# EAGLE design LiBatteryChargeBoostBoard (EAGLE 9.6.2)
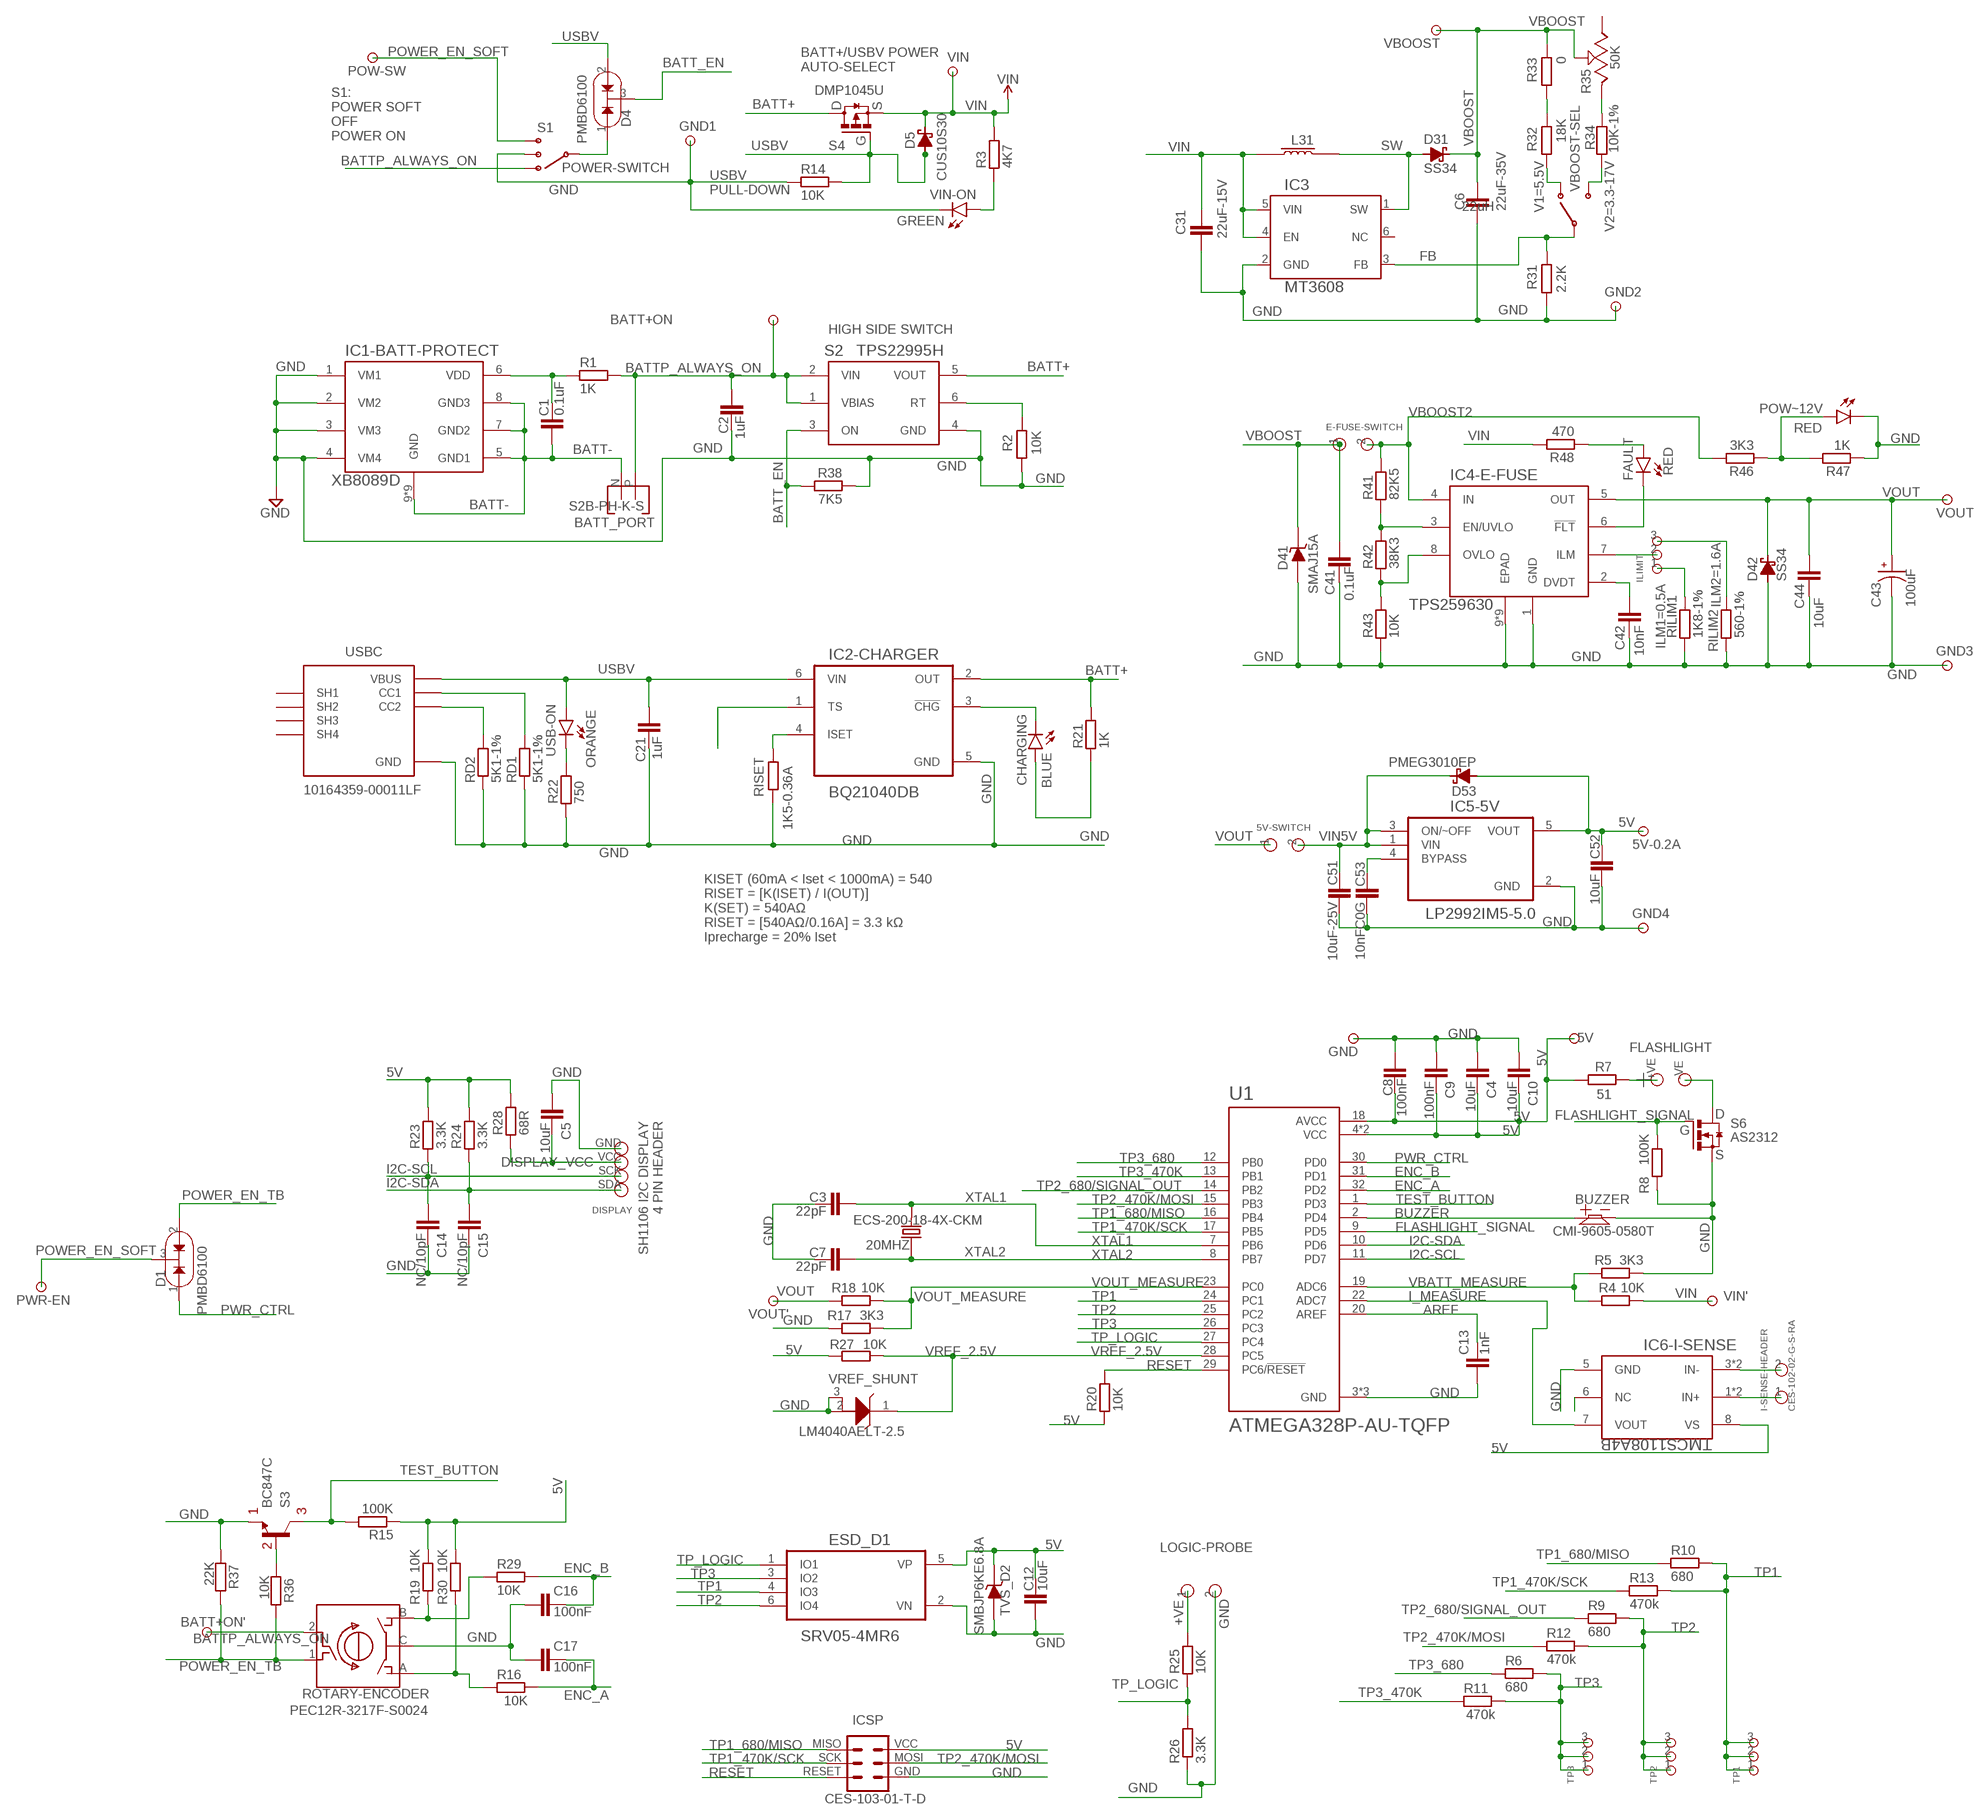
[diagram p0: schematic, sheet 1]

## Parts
5V  TEST-POINT-TH  [TEST-POINT-TH-1MM]
5V-0.2A  TEST-POINT-TH  [TEST-POINT-TH-1MM]
5V-SWITCH  HEADER-2PIN-0.1"P  [HEADER-2PIN-0.1"P]
20MHZ  ECS-200-18-4X-CKM  CRYSTAL-20MHZ-ECS-200-18-4X-CKM  [XTAL_ECS-200-18-4X-CKM]
BATT+ON  TEST-POINT-TH  [TEST-POINT-TH-1MM]
BATT+ON'  TEST-POINT-TH  [TEST-POINT-TH-1MM]
BATT_PORT  S2B-PH-K-S  [S2B-PH-K-S]
BUZZER  CMI-9605-0580T  BUZZER-ACTIVE-CMI-9605-0580T  [BUZZER-ACTIVE-CMI-9605-0580T]
C1  0.1uF  CAPACITOR_SMD0603  [0603]
C2  1uF  CAPACITOR_SMD0603  [0603]
C3  22pF  CAPACITOR_SMD0603  [0603]
C4  10uF  CAPACITOR_SMD0603  [0603]
C5  10uF  CAPACITOR1206  [1206]
C6  22uF-35V  CAPACITOR_SMD1206  [1206]
C7  22pF  CAPACITOR_SMD0603  [0603]
C8  100nF  CAPACITOR_SMD0603  [0603]
C9  100nF  CAPACITOR_SMD0603  [0603]
C10  10uF  CAPACITOR_SMD0603  [0603]
C12  10uF  CAPACITOR_SMD0603  [0603]
C13  1nF  CAPACITOR_SMD0603  [0603]
C14  NC/10pF  CAPACITOR_SMD0603  [0603]
C15  NC/10pF  CAPACITOR_SMD0603  [0603]
C16  100nF  CAPACITOR_SMD0603  [0603]
C17  100nF  CAPACITOR_SMD0603  [0603]
C21  1uF  CAPACITOR_SMD0603  [0603]
C31  22uF-15V  CAPACITOR_SMD1206  [1206]
C41  0.1uF  CAPACITOR_SMD0603  [0603]
C42  10nF  CAPACITOR_SMD0603  [0603]
C43  100uF  EEEFN1E101UP  [CAP_EEEFN1E101UP]
C44  10uF  CAPACITOR_SMD0603  [0603]
C51  10uF-25V  CAPACITOR0603  [0603]
C52  10uF  CAPACITOR0603  [0603]
C53  10nFC0G  CAPACITOR_SMD0603  [0603]
CHARGING  BLUE  LED0603  [0603-DIODE]
D1  PMBD6100  DIODE-DOUBLE-COMMON-CATHODE-PMBD6100,215  [SOT-23-3]
D4  PMBD6100  DIODE-DOUBLE-COMMON-CATHODE-PMBD6100,215  [SOT-23-3]
D5  CUS10S30  DIODE-SCHOTTKY-CUS10S30,H3F  [SOD-323]
D31  SS34  DIODE-SCHOTTKY-SS34  [SMA]
D41  SMAJ15A  DIODE-TVS-SMA  [SMA]
D42  SS34  DIODE-SCHOTTKY-SS34  [SMA]
D53  PMEG3010EP  DIODE-SCHOTTKY-PMEG3010EP,115  [SOD-128]
DISPLAY  DISPLAY-1.3"-SH1106-I2C  [DISPLAY-1.3"-SH1106-I2C]
E-FUSE-SWITCH  HEADER-2PIN-0.1"P  [HEADER-2PIN-0.1"P]
ESD_D1  SRV05-4MR6  SRV05-4MR6T1G  [SOT-23-6]
FAULT  RED  LED0603  [0603-DIODE]
FLASHLIGHT  HEADER-2PIN-0.2"P  [HEADER-2PIN-0.2"P]
GND  TEST-POINT-TH  [TEST-POINT-TH-1MM]
GND1  TEST-POINT-TH  [TEST-POINT-TH-1MM]
GND2  TEST-POINT-TH  [TEST-POINT-TH-1MM]
GND3  TEST-POINT-TH  [TEST-POINT-TH-1MM]
GND4  TEST-POINT-TH  [TEST-POINT-TH-1MM]
I-SENSE-HEADER  CES-102-02-G-S-RA  HEADER-2PIN-0.1"P  [HEADER-2PIN-0.1"P]
IC1-BATT-PROTECT  XB8089D  [SOIC-8-POWER-PAD]
IC2-CHARGER  BQ21040DB  BQ21040DBVR  [SOT-23-6]
IC3  MT3608  [SOT-23-6]
IC4-E-FUSE  TPS259630  TPS259621DDAR  [SOIC-8-POWER-PAD]
IC5-5V  LP2992IM5-5.0  [SOT-23-5]
IC6-I-SENSE  TMCS1108A4B  TMCS1108A4B-CURRENT-SENSE  [SOIC-8]
ICSP  CES-103-01-T-D  HEADER-ICSP-0.1"P  [HEADER-ICSP-0.1"P]
ILIMIT  HEADER-3PIN-0.1"P  [HEADER-3PIN-0.1"P]
L31  22uH  INDUCTOR-SMRH74-220MT  [INDUCTOR-SMRH74-220MT]
LOGIC-PROBE  HEADER-2PIN-0.1"P  [HEADER-2PIN-0.1"P]
POW-SW  TEST-POINT-TH  [TEST-POINT-TH-1MM]
POW~12V  RED  LED1206  [1206-DIODE]
PWR-EN  TEST-POINT-TH  [TEST-POINT-TH-1MM]
R1  1K  RESISTOR_SMD0603  [0603]
R2  10K  RESISTOR_SMD0603  [0603]
R3  4K7  RESISTOR_SMD0603  [0603]
R4  10K  RESISTOR_SMD0603  [0603]
R5  3K3  RESISTOR_SMD0603  [0603]
R6  680  RESISTOR_SMD1206  [1206]
R7  51  RESISTOR_SMD1206  [1206]
R8  100K  RESISTOR_SMD0603  [0603]
R9  680  RESISTOR_SMD1206  [1206]
R10  680  RESISTOR_SMD1206  [1206]
R11  470k  RESISTOR_SMD1206  [1206]
R12  470k  RESISTOR_SMD1206  [1206]
R13  470k  RESISTOR_SMD1206  [1206]
R14  10K  RESISTOR_SMD0603  [0603]
R15  100K  RESISTOR_SMD0603  [0603]
R16  10K  RESISTOR_SMD0603  [0603]
R17  3K3  RESISTOR_SMD0603  [0603]
R18  10K  RESISTOR_SMD0603  [0603]
R19  10K  RESISTOR_SMD0603  [0603]
R20  10K  RESISTOR_SMD0603  [0603]
R21  1K  RESISTOR_SMD0603  [0603]
R22  750  RESISTOR_SMD0603  [0603]
R23  3.3K  RESISTOR_SMD0603  [0603]
R24  3.3K  RESISTOR_SMD0603  [0603]
R25  10K  RESISTOR_SMD0603  [0603]
R26  3.3K  RESISTOR_SMD0603  [0603]
R27  10K  RESISTOR_SMD0603  [0603]
R28  68R  RESISTOR_SMD0603  [0603]
R29  10K  RESISTOR_SMD0603  [0603]
R30  10K  RESISTOR_SMD0603  [0603]
R31  2.2K  RESISTOR_SMD0603  [0603]
R32  18K  RESISTOR_SMD0603  [0603]
R33  0  RESISTOR_SMD0603  [0603]
R34  10K-1%  RESISTOR_SMD0603  [0603]
R35  50K  ROTARY-POTENTIOMETER-3386P-1-503TLF  [ROTARY-POTENTIOMETER-3386P]
R36  10K  RESISTOR_SMD0603  [0603]
R37  22K  RESISTOR_SMD0603  [0603]
R38  7K5  RESISTOR_SMD0603  [0603]
R41  82K5  RESISTOR_SMD0603  [0603]
R42  38K3  RESISTOR_SMD0603  [0603]
R43  10K  RESISTOR_SMD0603  [0603]
R46  3K3  RESISTOR_SMD0603  [0603]
R47  1K  RESISTOR_SMD0603  [0603]
R48  470  RESISTOR_SMD0603  [0603]
RD1  5K1-1%  RESISTOR_SMD0603  [0603]
RD2  5K1-1%  RESISTOR_SMD0603  [0603]
RILIM1  1K8-1%  RESISTOR_SMD0603  [0603]
RILIM2  560-1%  RESISTOR_SMD0603  [0603]
RISET  1K5-0.36A  RESISTOR_SMD0603  [0603]
ROTARY-ENCODER  PEC12R-3217F-S0024  [PEC12R-3217F-S0024]
S1  POWER-SWITCH  SLIDE-SWITCH-SP3T-VER-TH-MINI  [CSS-1310MC]
S2  TPS22995H  TPS22995H-Q1  [SOT-23-6]
S3  BC847C  [SOT-23-3]
S4  DMP1045U  [SOT-23-3]
S6  AS2312  AS2312AS2312  [SOT-23-3]
TP1  HEADER-3PIN-0.1"P  [HEADER-3PIN-0.1"P]
TP2  HEADER-3PIN-0.1"P  [HEADER-3PIN-0.1"P]
TP3  HEADER-3PIN-0.1"P  [HEADER-3PIN-0.1"P]
TVS_D2  SMBJP6KE6.8A  SMBJP6KE6.8A-TP  [DIOM5336X244N]
U1  ATMEGA328P-AU-TQFP  [TQFP32]
USB-ON  ORANGE  LED0603  [0603-DIODE]
USBC  10164359-00011LF  USB-C-RECEPTABLE-10164359-00011LF  [USB-C-RECEPTABLE-1016435900011LF]
VBOOST  TEST-POINT-TH  [TEST-POINT-TH-1MM]
VBOOST-SEL  SLIDE-SWITCH-SPDT-VERTICLE-TH  [SLW-883935-2A-D]
VIN  TEST-POINT-TH  [TEST-POINT-TH-1MM]
VIN'  TEST-POINT-TH  [TEST-POINT-TH-1MM]
VIN-ON  GREEN  LED0603  [0603-DIODE]
VOUT  TEST-POINT-TH  [TEST-POINT-TH-1MM]
VOUT'  TEST-POINT-TH  [TEST-POINT-TH-1MM]
VREF_SHUNT  LM4040AELT-2.5  LM4040AELT-2.5-SOT23  [SOT-23-3]

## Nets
5V: 5V-0.2A.P$1 5V.P$1 C4.1 C8.2 C9.1 C10.1 C12.1 C52.2 D53.A ESD_D1.5(VP) IC5-5V.5(VOUT) IC6-I-SENSE.8(VS) ICSP.VCC R7.1 R15.1 R19.2 R20.1 R23.2 R24.2 R27.1 R28.2 R30.2 TVS_D2.C U1.4(VCC) U1.6(VCC) U1.18(AVCC)
!FLT: FAULT.C IC4-E-FUSE.6(!FLT)
+VE: LOGIC-PROBE.1 R25.2
A: R16.1 R30.1 ROTARY-ENCODER.A
AREF: C13.1 U1.20(AREF)
B: R19.1 R29.1 ROTARY-ENCODER.B
BATT+: IC2-CHARGER.2(OUT) R21.2 S2.5(VOUT) S4.3(D)
BATT-: BATT_PORT.N C1.2 IC1-BATT-PROTECT.5(GND1) IC1-BATT-PROTECT.7(GND2) IC1-BATT-PROTECT.8(GND3) IC1-BATT-PROTECT.9(GND) IC1-BATT-PROTECT.10(GND) IC1-BATT-PROTECT.11(GND) IC1-BATT-PROTECT.12(GND) IC1-BATT-PROTECT.13(GND) IC1-BATT-PROTECT.14(GND) IC1-BATT-PROTECT.15(GND) IC1-BATT-PROTECT.16(GND) IC1-BATT-PROTECT.17(GND)
BATT_EN: D4.3(C) R38.2 S2.3(ON)
BATTP_ALWAYS_ON: BATT+ON'.P$1 BATT+ON.P$1 BATT_PORT.P C2.2 R1.2 ROTARY-ENCODER.2 S1.1 S2.1(VBIAS) S2.2(VIN)
BJT-B: R36.1 S3.1(B)
BUZZER: BUZZER.P$1 U1.2(PD4)
BYP1: C53.2 IC5-5V.4(BYPASS)
CHG: CHARGING.C IC2-CHARGER.3(!CHG)
DISPLAY_VCC: C5.1 DISPLAY.VCC R28.1
DVDT: C42.2 IC4-E-FUSE.2(DVDT)
EN/UVLO: IC4-E-FUSE.3(EN/UVLO) R41.1 R42.2
ENC_A: C17.1 R16.2 U1.32(PD2)
ENC_B: C16.1 R29.2 U1.31(PD1)
FB: IC3.3(FB) R31.1 VBOOST-SEL.C
FL+: FLASHLIGHT.+VE R7.2
FL-: FLASHLIGHT.-VE S6.3(D)
FLASHLIGHT_SIGNAL: R8.1 S6.1(G) U1.9(PD5)
GND: BUZZER.P$2 C2.1 C3.1 C4.2 C5.2 C6.1 C7.1 C8.1 C9.2 C10.2 C12.2 C13.2 C14.1 C15.1 C16.2 C17.2 C21.1 C31.1 C41.1 C42.1 C43.2 C44.1 C51.1 C52.1 C53.1 D41.A D42.A DISPLAY.GND ESD_D1.2(VN) GND1.P$1 GND2.P$1 GND3.P$1 GND4.P$1 GND.P$1 IC1-BATT-PROTECT.1(VM1) IC1-BATT-PROTECT.2(VM2) IC1-BATT-PROTECT.3(VM3) IC1-BATT-PROTECT.4(VM4) IC2-CHARGER.5(GND) IC3.2(GND) IC4-E-FUSE.1(GND) IC4-E-FUSE.9(EPAD) IC4-E-FUSE.10(EPAD) IC4-E-FUSE.11(EPAD) IC4-E-FUSE.12(EPAD) IC4-E-FUSE.13(EPAD) IC4-E-FUSE.14(EPAD) IC4-E-FUSE.15(EPAD) IC4-E-FUSE.16(EPAD) IC4-E-FUSE.17(EPAD) IC5-5V.2(GND) IC6-I-SENSE.5(GND) ICSP.GND LOGIC-PROBE.2 POW~12V.C R2.2 R5.2 R8.2 R14.1 R17.1 R22.1 R26.1 R31.2 R37.1 R38.1 R43.1 R47.1 RD1.1 RD2.1 RILIM1.1 RILIM2.1 RISET.2 ROTARY-ENCODER.C S1.2 S2.4(GND) S3.2(E) S6.2(S) TVS_D2.A U1.3(GND) U1.5(GND) U1.21(GND) USBC.A12(GND) USBC.B12(GND) VIN-ON.C VREF_SHUNT.2(A) VREF_SHUNT.3(NC/A)
I2C-SCL: C14.2 DISPLAY.SCK R23.1 U1.11(PD7)
I2C-SDA: C15.2 DISPLAY.SDA R24.1 U1.10(PD6)
I_MEASURE: IC6-I-SENSE.7(VOUT) U1.22(ADC7)
ILM: IC4-E-FUSE.7(ILM) ILIMIT.2
ILM1: ILIMIT.1 RILIM1.2
ILM2: ILIMIT.3 RILIM2.2
IN+: I-SENSE-HEADER.1 IC6-I-SENSE.1(IN+) IC6-I-SENSE.2(IN+)
IN-: I-SENSE-HEADER.2 IC6-I-SENSE.3(IN-) IC6-I-SENSE.4(IN-)
ISET: IC2-CHARGER.4(ISET) RISET.1
N$1: RD2.2 USBC.B5(CC2)
N$2: RD1.2 USBC.A5(CC1)
N$3: R22.2 USB-ON.C
N$4: R32.2 VBOOST-SEL.1
N$5: R3.1 VIN-ON.A
N$7: FAULT.A R48.1
N$10: CHARGING.A R21.1
N$12: R32.1 R33.2
N$13: R34.2 VBOOST-SEL.2
N$18: POW~12V.A R46.1 R47.2
N$21: R34.1 R35.3(CCW)
NC: IC6-I-SENSE.6(NC)
OVLO: IC4-E-FUSE.8(OVLO) R42.1 R43.2
POWER_EN_SOFT: D1.3(C) POW-SW.P$1 PWR-EN.P$1 S1.3
POWER_EN_TB: D1.2(A2) R36.2 R37.2 ROTARY-ENCODER.1
PWR_CTRL: D1.1(A1) U1.30(PD0)
PWR_SW: D4.1(A1) S1.C
RESET: ICSP.RESET R20.2 U1.29(PC6/!RESET)
RT: R2.1 S2.6(RT)
SW: D31.A IC3.1(SW) L31.P$2
TEST_BUTTON: R15.2 S3.3(C) U1.1(PD3)
TP1: ESD_D1.4(IO3) R10.2 R13.2 TP1.1 TP1.2 TP1.3 U1.24(PC1)
TP1_470K/SCK: ICSP.SCK R13.1 U1.17(PB5)
TP1_680/MISO: ICSP.MISO R10.1 U1.16(PB4)
TP2: ESD_D1.6(IO4) R9.2 R12.2 TP2.1 TP2.2 TP2.3 U1.25(PC2)
TP2_470K/MOSI: ICSP.MOSI R12.1 U1.15(PB3)
TP2_680/SIGNAL_OUT: R9.1 U1.14(PB2)
TP3: ESD_D1.3(IO2) R6.2 R11.2 TP3.1 TP3.2 TP3.3 U1.26(PC3)
TP3_470K: R11.1 U1.13(PB1)
TP3_680: R6.1 U1.12(PB0)
TP_LOGIC: ESD_D1.1(IO1) R25.1 R26.2 U1.27(PC4)
TS: IC2-CHARGER.1(TS)
USBV: C21.2 D4.2(A2) D5.A IC2-CHARGER.6(VIN) R14.2 S4.1(G) USB-ON.A USBC.A9(VBUS) USBC.B9(VBUS)
VBATT_MEASURE: R4.2 R5.1 U1.19(ADC6)
VBOOST: C6.2 C41.2 D31.C D41.C E-FUSE-SWITCH.1 R33.1 R35.2(S) VBOOST.P$1
VBOOST2: E-FUSE-SWITCH.2 IC4-E-FUSE.4(IN) R41.2 R46.2
VDD: C1.1 IC1-BATT-PROTECT.6(VDD) R1.1
VIN: C31.2 D5.C IC3.4(EN) IC3.5(VIN) L31.P$1 R3.2 R4.1 R48.2 S4.2(S) VIN'.P$1 VIN.P$1
VIN5V: 5V-SWITCH.2 C51.2 D53.K(C) IC5-5V.1(VIN) IC5-5V.3(ON/~OFF)
VOUT: 5V-SWITCH.1 C43.1 C44.2 D42.C IC4-E-FUSE.5(OUT) R18.2 VOUT'.P$1 VOUT.P$1
VOUT_MEASURE: R17.2 R18.1 U1.23(PC0)
VREF_2.5V: R27.2 U1.28(PC5) VREF_SHUNT.1(C)
XTAL1: 20MHZ.2 C3.2 U1.7(PB6)
XTAL2: 20MHZ.1 C7.2 U1.8(PB7)
Unconnected: IC3.6(NC) R35.1(CW) USBC.SH1 USBC.SH2 USBC.SH3 USBC.SH4

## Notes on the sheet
- BATT+/USBV POWER
  AUTO-SELECT
- S1:
  POWER SOFT
  OFF
  POWER ON
- USBV
  PULL-DOWN
- V1=5.5V
- V2=3.3-17V
- HIGH SIDE SWITCH
- ILM2=1.6A
- ILM1=0.5A
- KISET (60mA < Iset < 1000mA) = 540
  RISET = [K(ISET) / I(OUT)] 
  K(SET) = 540AΩ
  RISET = [540AΩ/0.16A] = 3.3 kΩ
  Iprecharge = 20% Iset

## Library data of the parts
5V 5V-0.2A BATT+ON BATT+ON' GND GND1-GND4 POW-SW PWR-EN VBOOST VIN VIN' VOUT VOUT' = .MyComponents:TEST-POINT: TEST POINT
5V-SWITCH E-FUSE-SWITCH I-SENSE-HEADER LOGIC-PROBE = .MyComponents:HEADER-2PIN-0.1"P
20MHZ = .MyComponents:CRYSTAL-20MHZ-ECS-200-18-4X-CKM: 20MHz Crystal Check availability; AVAILABILITY: In Stock; CHECK_PRICES: https://www.snapeda.com/parts/ECS-200-18-4X-CKM/ECS+Inc./view-part/?ref=eda; DATASHEET: https://ecsxtal.com/store/pdf/hc-49usx.pdf; DESCRIPTION: 20 MHz ±10ppm Crystal 18pF 30 Ohms HC-49/US; MF: ECS Inc.; MP: ECS-200-18-4X-CKM; PACKAGE: HC-49US ECS Inc.; PRICE: None; PURCHASE-URL: https://www.snapeda.com/api/url_track_click_mouser/?unipart_id=5049327&manufacturer=ECS Inc.&part_name=ECS-200-18-4X-CKM&search_term=None; SNAPEDA_LINK: https://www.snapeda.com/parts/ECS-200-18-4X-CKM/ECS+Inc./view-part/?ref=snap
BATT_PORT = .MyComponents:S2B-PH-K-S: S2B-PH-K-S
BUZZER = .MyComponents:BUZZER-ACTIVE-CMI-9605-0580T: Active Buzzer WST-0905T; DATASHEET: https://www.mouser.com/datasheet/2/670/cmi_9605_0580t-1776530.pdf
C1-C4 C6-C10 C12-C17 C21 C31 C41 C42 C44 C53 = .MyComponents:CAPACITOR_SMD: capacitor 1206
C5 = .MyComponents:CAPACITOR1206: capacitor 1206
C43 = .MyComponents:EEEFN1E101UP: Check availability; AVAILABILITY: In Stock; CHECK_PRICES: https://www.snapeda.com/parts/EEE-FN1E101UP/Panasonic/view-part/?ref=eda; DESCRIPTION: Capacitor,25VDC, 100uF,SMD'Electrolytic | Panasonic Electronic Components EEE-FN1E101UP; MF: Panasonic Electronic Components; MP: EEE-FN1E101UP; PACKAGE: RADIAL-2 Panasonic; PRICE: None; PURCHASE-URL: https://www.snapeda.com/api/url_track_click_mouser/?unipart_id=6178105&manufacturer=Panasonic Electronic Components&part_name=EEE-FN1E101UP&search_term=eee-fn1e101up; SNAPEDA_LINK: https://www.snapeda.com/parts/EEE-FN1E101UP/Panasonic/view-part/?ref=snap
C51 C52 = .MyComponents:CAPACITOR0603: capacitor 0603
CHARGING FAULT POW~12V USB-ON VIN-ON = .MyComponents:LED
D1 D4 = .MyComponents:DIODE-DOUBLE-COMMON-CATHODE-PMBD6100,215: Dual diode common cathode Mouser Datasheet single diode loaded − 215 mA double diode loaded − 125 mA continuous reverse voltage − 70 V repetitive peak reverse voltage − 85 V IFRM repetitive peak forward current − 450 mA IFSM non-repetitive peak forward current square wave; Tj = 25 °C prior to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; DATASHEET: https://www.mouser.com/datasheet/2/916/PMBD6100-2938376.pdf; VALUE: PMBD6100,215
D5 = .MyComponents:DIODE-SCHOTTKY-CUS10S30,H3F: CUS10S30,H3F
D31 D42 = .MyComponents:DIODE-SCHOTTKY-SS34: Part Number: SS34 / Forward Current : 3 A / Maxixum Repetitive Peak Reverse Voltage : 40 V
D41 = .MyComponents:DIODE-TVS-
D53 = .MyComponents:DIODE-SCHOTTKY-PMEG3010EP,115: Diode 30 V 1A Surface Mount SOD-128/CFP5
DISPLAY = .MyComponents:DISPLAY-1.3"-SH1106-I2C: SH1106 I2C DISPLAY https://www.amazon.com/dp/B0C3L54TL6
ESD_D1 = .MyComponents:SRV05-4MR6T1G: ESD Circuit Protection 17.5V Clamp 5A (8/20µs) Ipp Tvs Diode Surface Mount 6-TSOP DigiKey Check availability; AVAILABILITY: In Stock; CHECK_PRICES: https://www.snapeda.com/parts/SRV05-4MR6T1G/Onsemi/view-part/?ref=eda; DESCRIPTION: 17.5V Clamp 5A (8/20µs) Ipp Tvs Diode Surface Mount 6-TSOP; MF: ON Semiconductor; MP: SRV05-4MR6T1G; PACKAGE: TSOP-6 ON Semiconductor; PRICE: None; PURCHASE-URL: https://www.snapeda.com/api/url_track_click_mouser/?unipart_id=95760&manufacturer=ON Semiconductor&part_name=SRV05-4MR6T1G&search_term=None; SNAPEDA_LINK: https://www.snapeda.com/parts/SRV05-4MR6T1G/Onsemi/view-part/?ref=snap
FLASHLIGHT = .MyComponents:HEADER-2PIN-0.2"P: 5MM 2 PIN HEADER
IC1-BATT-PROTECT = .MyComponents:XB8089D: XB8089D One Cell Lithium-ion/Polymer Battery Protection IC datasheet FEATURES ·Protection of Charger Reverse Connection ·Protection of Battery Cell Reverse Connection ·Integrate Advanced Power MOSFET with Equivalent of 20mΩ RSS(ON) ·SOP8-PP Package ·Only One External Capacitor Required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
IC2-CHARGER = .MyComponents:BQ21040DBVR: battery charger Check Availability; AVAILABILITY: In Stock; CHECK_PRICES: https://www.snapeda.com/parts/BQ21040DBVR/Texas+Instruments/view-part/?ref=eda; DESCRIPTION: 1-cell, 0.8-A Li-ion and Li-polymer battery charger; MF: Texas Instruments; MP: BQ21040DBVR; PACKAGE: SOT-23-6 Texas Instruments; PRICE: None; PURCHASE-URL: https://www.snapeda.com/api/url_track_click_mouser/?unipart_id=505197&manufacturer=Texas Instruments&part_name=BQ21040DBVR&search_term=bq21040dbvr; SNAPEDA_LINK: https://www.snapeda.com/parts/BQ21040DBVR/Texas+Instruments/view-part/?ref=snap
IC3 = .MyComponents:MT3608: High Efficiency 1.2MHz 2A Step Up Converter datasheet Circuit • Integrated 80mΩ Power MOSFET • 2V to 24V Input Voltage • 1.2MHz Fixed Switching Frequency • Internal 4A Switch Current Limit • Adjustable Output Voltage • Internal Compensation • Up to 28V Output Voltage • Automatic Pulse Frequency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
IC4-E-FUSE = .MyComponents:TPS259621DDAR: Electronic Fuse Regulator 2A 8-SO PowerPad Texas Instruments TPS259621DDAR The TPS2596xx family of eFuses (integrated FET hot-swap devices) is a highly integrated circuit protection and power management solution in a small package. datasheet DigiKey
IC5-5V = .MyComponents:LP2992IM5-5.0: LP2992 Micropower 250-mA Low-Noise Ultra-Low-Dropout Regulator in SOT-23 and WSON Packages Designed for Use With Very Low-ESR Output Capacitors Datasheet DigiKey Input Voltage Range: 2.2 V to 16 V Output Voltage Range: 1.5 V to 5 V Output Voltage Accuracy 1% (A Grade); AVAILABILITY: In Stock; CHECK_PRICES: https://www.snapeda.com/parts/LP2992IM5-5.0/NOPB/Texas+Instruments/view-part/?ref=eda; DESCRIPTION: 250-mA, 16-V, low-dropout voltage regulator with enable; MF: Texas Instruments; MP: LP2992IM5-5.0/NOPB; PACKAGE: SOT-23-5 Texas Instruments; PRICE: None; PURCHASE-URL: https://www.snapeda.com/api/url_track_click_mouser/?unipart_id=26545&manufacturer=Texas Instruments&part_name=LP2992IM5-5.0/NOPB&search_term=lp2992im5-5.0/nopb; SNAPEDA_LINK: https://www.snapeda.com/parts/LP2992IM5-5.0/NOPB/Texas+Instruments/view-part/?ref=snap
IC6-I-SENSE = .MyComponents:TMCS1108A4B-CURRENT-SENSE: TMCS1108A4BQDR Current Sensor 1 Channel Hall Effect Bidirectional 8-SOIC (0.154", 3.90mm Width) DigiKey Datasheet
ICSP = .MyComponents:HEADER-ICSP-0.1"P: ISP HEADER 2X3 2.54MM
ILIMIT TP1-TP3 = .MyComponents:HEADER-3PIN-0.1"P
L31 = .MyComponents:INDUCTOR-SMRH74-220MT: 22uH Inductor +-20%
R1-R34 R36-R38 R41-R43 R46-R48 RD1 RD2 RILIM1 RILIM2 RISET = .MyComponents:RESISTOR_SMD: resistor smd
R35 = .MyComponents:ROTARY-POTENTIOMETER-: 50 kOhms 0.5W, 1/2W PC Pins Through Hole Trimmer Potentiometer Cermet 1.0 Turn Top Finger Adjustment DigiKey
ROTARY-ENCODER = .MyComponents:PEC12R-3217F-S0024: Rotary Encoder with Push Button and Bushing Bourns Inc digikey
S1 = .MyComponents:SLIDE-SWITCH-SP3T-: CUI Devices Slide Switch SP3T SLW-1516255-6A-RA-D Right Angle TH
S2 = .MyComponents:TPS22995H-Q1: 5.5-V, 3-A, 19-mΩ On-Resistance Automotive Load Switch DigiKey • Input operating voltage range (VIN): 0.8 V–5.5 V • Bias voltage supply (VBIAS): 1.5 V–5.5 V • Maximum continuous current: 3 A • ON-resistance (RON): 19 mΩ (typ.) • Adjustable slew rate control through external resistor • Quick Output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
S3 = .MyComponents:BC847C: BC847C Bipolar (BJT) Transistor NPN 45 V 100 mA 300MHz 200 mW Surface Mount SOT-23 https://www.digikey.com/en/products/detail/good-ark-semiconductor/BC847C/18648944
S4 = .MyComponents:DMP1045U: DMP1045U PMOSFET SOT-23-3 VDSS -12V RDS(ON) Max ID 31mΩ @ VGS = -4.5V 5.2A 45mΩ @ VGS =-2.5V 4.3A ON CHARACTERISTICS Gate Threshold Voltage VGS(TH) -0.3 -0.55 -1.0 V Diode Forward Voltage VSD — -0.6 — V ABSOLUTE MAXIMUM RATINGS (@TA = +25°C, unless otherwise specified.) Characteristic Symbol Value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
S6 = .MyComponents:AS2312: AS2312 N-Channel 20 V 6.8A (Ta) 1.2W (Ta) Surface Mount SOT-23 https://www.digikey.com/en/products/detail/anbon-semiconductor-int-l-limited/AS2312/16708465
TVS_D2 = .MyComponents:SMBJP6KE6.8A-TP: SMBJ Series 600 W 6.8 V Uni-Directional Surface Mount TVS Diode - SMB; CHECK_PRICES: https://www.snapeda.com/parts/SMBJP6KE6.8A-TP/Micro+Commercial+Components/view-part/?ref=eda; DESCRIPTION: 10.5V Clamp 58.1A Ipp Tvs Diode Surface Mount DO-214AA (SMBJ); DIGIKEY_PART_NUMBER: SMBJP6KE6.8A-TPMSTR-ND; MF: Micro Commercial; MP: SMBJP6KE6.8A-TP; PACKAGE: DO-214 MCC; PURCHASE-URL: https://www.snapeda.com/api/url_track_click_mouser/?unipart_id=577204&manufacturer=Micro Commercial&part_name=SMBJP6KE6.8A-TP&search_term=smbjp6ke6.8a; SNAPEDA_LINK: https://www.snapeda.com/parts/SMBJP6KE6.8A-TP/Micro+Commercial+Components/view-part/?ref=snap
U1 = .MyComponents:ATMEGA328P-AU-TQFP: Check availability; AVAILABILITY: In Stock; CHECK_PRICES: https://www.snapeda.com/parts/ATMEGA328P-AU/Microchip/view-part/?ref=eda; DESCRIPTION: AVR AVR® ATmega Microcontroller IC 8-Bit 20MHz 32KB (16K x 16) FLASH 32-TQFP (7x7); MF: Microchip; MP: ATMEGA328P-AU; PACKAGE: TQFP-32 Microchip; PRICE: None; PURCHASE-URL: https://www.snapeda.com/api/url_track_click_mouser/?unipart_id=44280&manufacturer=Microchip&part_name=ATMEGA328P-AU&search_term=atmega328p-au; SNAPEDA_LINK: https://www.snapeda.com/parts/ATMEGA328P-AU/Microchip/view-part/?ref=snap
USBC = .MyComponents:USB-C-RECEPTABLE-10164359-00011LF: USB-C (USB TYPE-C) Receptacle Connector 24 (6+18 Dummy) Position Surface Mount, Right Angle; Through Hole USB Type C Receptacle SMT Single Row 6Pin Source: Datasheet Check availability; AVAILABILITY: In Stock; CHECK_PRICES: https://www.snapeda.com/parts/10164359-00011LF/Amphenol/view-part/?ref=eda; DESCRIPTION: USB Type C Receptacle SMT Single Row 6Pin; MF: Amphenol FCI; MP: 10164359-00011LF; PACKAGE: None; PRICE: None; PURCHASE-URL: https://www.snapeda.com/api/url_track_click_mouser/?unipart_id=11778037&manufacturer=Amphenol FCI&part_name=10164359-00011LF&search_term=10164359-00011lf; SNAPEDA_LINK: https://www.snapeda.com/parts/10164359-00011LF/Amphenol/view-part/?ref=snap
VBOOST-SEL = .MyComponents:SLIDE-SWITCH-SPDT-: spdt slide switch SLW-883935-2A-D verticle th SLW-913535-2A-RA-D Right Angle Th
VREF_SHUNT = .MyComponents:LM4040AELT-2.5-SOT23: STMicroelectronics Shunt Voltage Reference IC Fixed 2.5V V ±0.1% 15 mA SOT-23-3 https://www.digikey.com/en/products/detail/stmicroelectronics/LM4040AELT-2-5/16184070 https://www.mouser.com/ProductDetail/511-LM4040AELT-2.5; DATASHEET: https://www.st.com/resource/en/datasheet/lm4040.pdf

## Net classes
0 default: clearance 0.205 mm

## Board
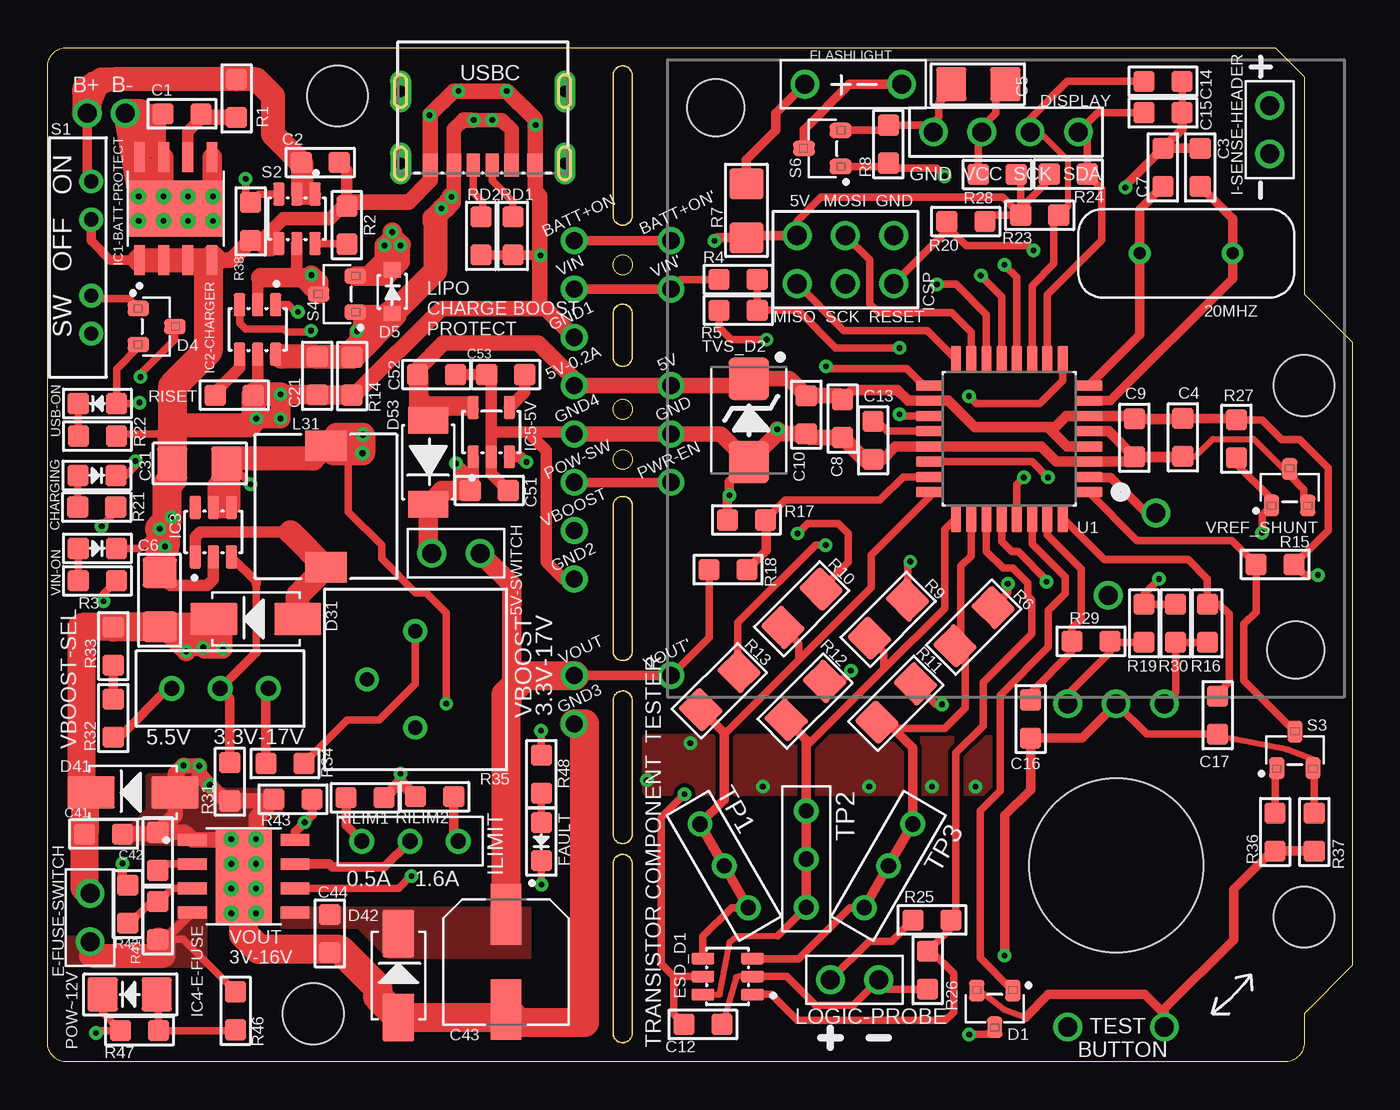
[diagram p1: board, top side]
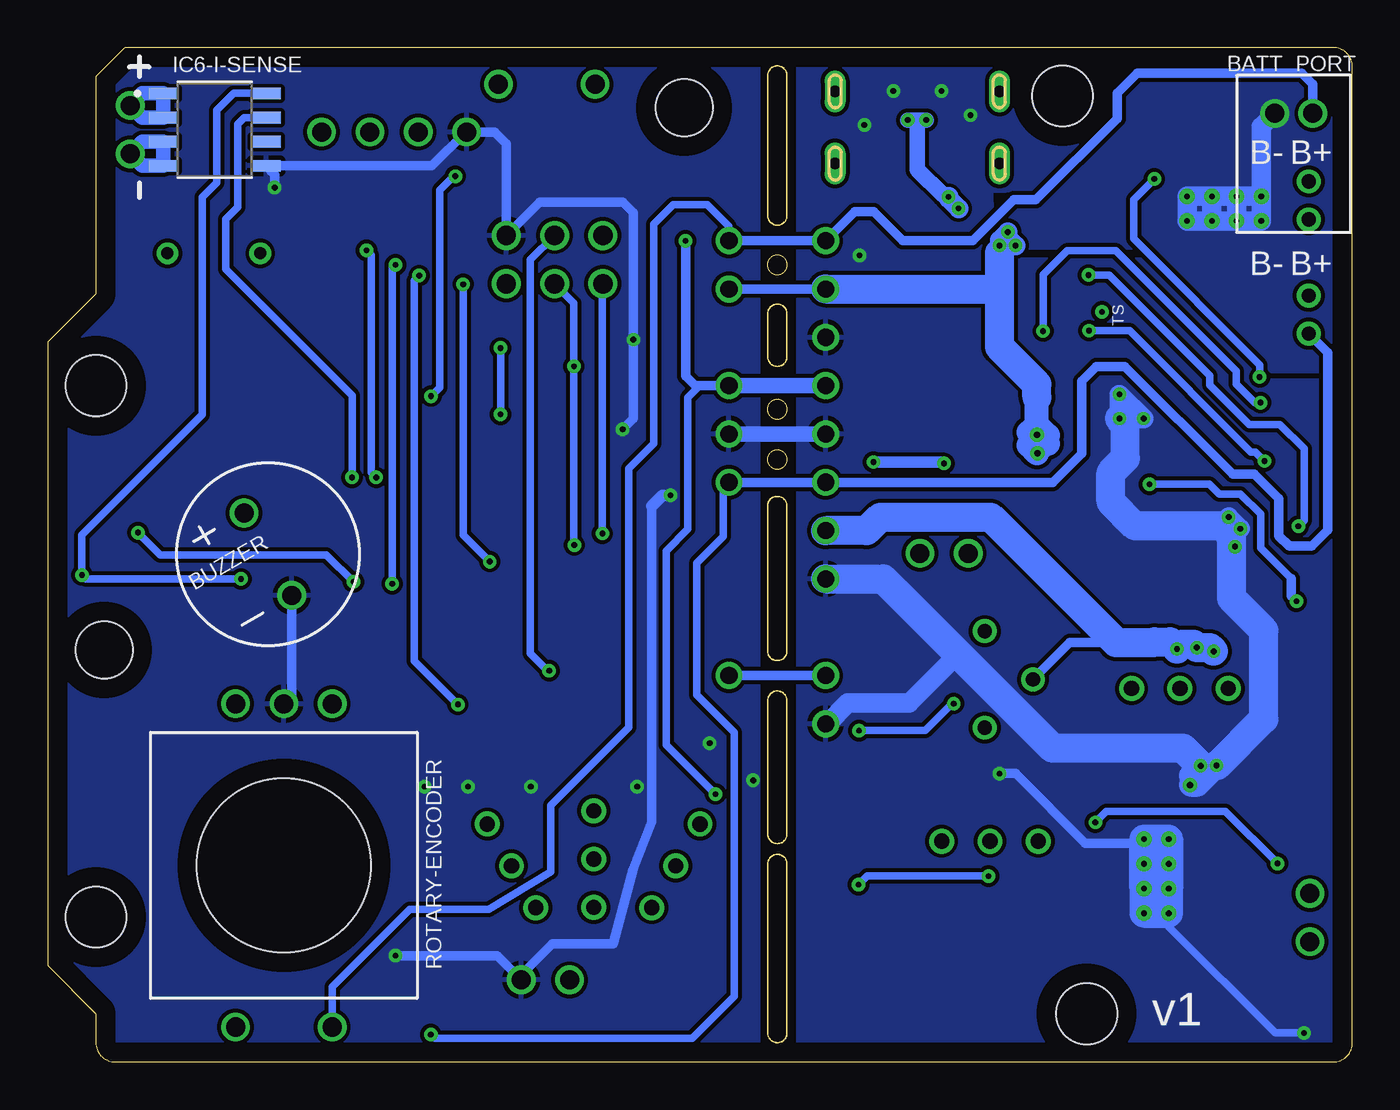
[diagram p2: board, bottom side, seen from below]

Size 68.58 x 53.34 mm. Coordinates in mm from the lower left corner, seen from the top.
Outline: 68.58,5.08 66.04,2.54 66.04,1.02 arc-90 65.02,0 1.02,0 arc-90 0,1.02 0,52.32 arc-90 1.02,53.34 64.52,53.34 66.04,51.82 66.04,40.39 68.58,37.85 68.58,5.08
Copper layers (1*16): Top 0.035mm / dielectric 1.5mm / Bottom 0.035mm
Design rules "default *": minimum track width 6mil, minimum drill 0.3mm, track to track 0.2mm, track to pad 0.2mm, pad to pad 0.2mm, via to via 10mil, smd to smd 0.2mm, copper to edge 40mil, drill to drill 0.5mm, minimum pad ring 10mil, minimum via ring 8mil, stop-mask expansion 4mil, vias tented up to drill 0mil, thermal gap 10mil
Holes 3.2 mm at 15.24,50.8 13.97,2.54 66.04,7.62 66.04,35.56
tKeepout: area 13.2,48.8 to 17.2,52.8; area 12,0.5 to 16,4.5; area 64,5.6 to 68,9.6; area 64,33.6 to 68,37.6
bKeepout: area 13.2,48.8 to 17.2,52.8; area 12,0.5 to 16,4.5; area 64,5.6 to 68,9.6; area 64,33.6 to 68,37.6
Milling: area 29.7,33.8 to 30.7,34.8; area 29.7,31.2 to 30.7,32.2; area 29.7,41.4 to 30.7,42.4; 30 lines

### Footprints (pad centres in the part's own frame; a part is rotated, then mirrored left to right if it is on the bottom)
TEST-POINT-TH-1MM = drill 0.9: P$1 0,0
HEADER-2PIN-0.1"P = drill 1: 1 -1.27,0; 2 1.27,0
XTAL_ECS-200-18-4X-CKM = drill 0.63 pad 1.03: 1 -2.44,0; 2 2.44,0
S2B-PH-K-S = drill 1: N 0.984,-2.54; P -1.016,-2.54
BUZZER-ACTIVE-CMI-9605-0580T = drill 1: P$1 0,2.5; P$2 0,-2.5
0603 = smd 1.1 x 1.1: 1 -1,0; 2 1,0
1206 = smd 1.6 x 1.803: 1 -1.422,0; 2 1.422,0
CAP_EEEFN1E101UP = smd 3.2 x 1.6: 1 -2.5,0; 2 2.5,0
0603-DIODE = smd 1.1 x 1.1: A 1,0; C -1,0
SOT-23-3 = smd 0.8 x 1.13: 1 -0.95,-0.96; 2 0.95,-0.96; 3 0,0.96
SOD-323 = smd 0.8 x 0.9: A -1.16,-0.03; C 1.14,-0.03
SMA = smd 2.5 x 1.7: A -2.205,0; C 2.205,0
SOD-128 = smd 1.4 x 2.1: A -2.11,-0.06; K 2.29,-0.06
DISPLAY-1.3"-SH1106-I2C = drill 1: GND -3.81,-1.27; SCK 1.27,-1.27; SDA 3.81,-1.27; VCC -1.27,-1.27 | hole 3: -15.24,0; 15.24,-28.5
SOT-23-6 = smd 1.2 x 0.6: 1 -1.3,0.95; 2 -1.3,0; 3 -1.3,-0.95; 4 1.3,-0.95; 5 1.3,0; 6 1.3,0.95
HEADER-2PIN-0.2"P = drill 1: +VE -2.54,0; -VE 2.54,0
SOIC-8-POWER-PAD = smd 1.55 x 0.6: 1 -2.7,1.905; 2 -2.7,0.635; 3 -2.7,-0.635; 4 -2.7,-1.905; 5 2.7,-1.905; 6 2.7,-0.635; 7 2.7,0.635; 8 2.7,1.905 | smd 2.95 x 4.9: 9 0,0 | drill 0.3: 10 -0.65,1.95; 11 0.65,1.95; 12 -0.65,0.65; 13 0.65,0.65; 14 -0.65,-0.65; 15 0.65,-0.65; 16 -0.65,-1.95; 17 0.65,-1.95
SOT-23-5 = smd 1.2 x 0.6: 1 -1.3,0.95; 2 -1.3,0; 3 -1.3,-0.95; 4 1.3,-0.95; 5 1.3,0.95
SOIC-8 = smd 1.55 x 0.6: 1 -2.7,1.905; 2 -2.7,0.635; 3 -2.7,-0.635; 4 -2.7,-1.905; 5 2.7,-1.905; 6 2.7,-0.635; 7 2.7,0.635; 8 2.7,1.905
HEADER-ICSP-0.1"P = drill 1.016: GND 2.54,1.27; MISO -2.54,-1.27; MOSI 0,1.27; RESET 2.54,-1.27; SCK 0,-1.27; VCC -2.54,1.27
HEADER-3PIN-0.1"P = drill 0.8: 1 -2.54,0; 2 0,0; 3 2.54,0
INDUCTOR-SMRH74-220MT = smd 2.2 x 1.6: P$1 0,3.2; P$2 0,-3.2
1206-DIODE = smd 1.6 x 1.803: A 1.422,0; C -1.422,0
ROTARY-POTENTIOMETER-3386P = drill 0.75: 1 2.54,0; 2 0,-2.54; 3 -2.54,0
PEC12R-3217F-S0024 = drill 1: 1 -2.54,8.5; 2 2.54,8.5; A -2.54,-8.5; B 2.54,-8.5; C 0,-8.5 | hole 9.144: 0,0
CSS-1310MC = drill 0.75: 1 -4,0; 2 -2,0; 3 4,0; C 2,0
DIOM5336X244N = smd 2.22 x 2.13: A 2.19,0; C -2.19,0
TQFP32 = smd 1.47 x 0.55: 1 -4.17,2.8; 2 -4.17,2; 3 -4.17,1.2; 4 -4.17,0.4; 5 -4.17,-0.4; 6 -4.17,-1.2; 7 -4.17,-2; 8 -4.17,-2.8; 17 4.17,-2.8; 18 4.17,-2; 19 4.17,-1.2; 20 4.17,-0.4; 21 4.17,0.4; 22 4.17,1.2; 23 4.17,2; 24 4.17,2.8 | smd 0.55 x 1.47: 9 -2.8,-4.17; 10 -2,-4.17; 11 -1.2,-4.17; 12 -0.4,-4.17; 13 0.4,-4.17; 14 1.2,-4.17; 15 2,-4.17; 16 2.8,-4.17; 25 2.8,4.17; 26 2,4.17; 27 1.2,4.17; 28 0.4,4.17; 29 -0.4,4.17; 30 -1.2,4.17; 31 -2,4.17; 32 -2.8,4.17
USB-C-RECEPTABLE-1016435900011LF = smd 0.7 x 1.2: A5 -0.5,3.03; B5 0.5,3.03 | smd 0.76 x 1.2: A9 1.52,3.03; B9 -1.52,3.03 | smd 0.8 x 1.2: A12 2.75,3.03; B12 -2.75,3.03 | drill 0.6 pad 1.1 long: SH1 -4.32,2.95; SH2 4.32,2.95; SH3 -4.32,-0.85; SH4 4.32,-0.85
SLW-883935-2A-D = drill 0.8: 1 -2.54,0; 2 2.54,0; C 0,0

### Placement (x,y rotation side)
5V  32.77,35.56 0 top
5V-0.2A  27.69,35.56 70 top
5V-SWITCH  21.46,26.75 180 top
20MHZ  59.84,42.52 0 top
BATT+ON  27.69,43.18 70 top
BATT+ON'  32.77,43.18 0 top
BATT_PORT  3.1,47.34 180 bottom
BUZZER  57,26.7 30 bottom
C1  7.07,49.85 180 top
C2  14.33,47.29 180 top
C3  60.58,47.04 270 top
C4  59.66,32.84 270 top
C5  48.92,51.41 180 top
C6  5.89,24.31 270 top
C7  58.62,47.04 270 top
C8  41.78,33.83 90 top
C9  57.12,32.82 270 top
C10  39.88,34.04 270 top
C12  34.44,1.98 0 top
C13  43.38,32.69 270 top
C14  58.62,51.56 180 top
C15  58.62,49.91 180 top
C16  51.66,18.03 270 top
C17  61.49,18.24 270 top
C21  14.17,36.08 90 top
C31  7.98,31.47 0 top
C41  2.95,11.99 180 top
C42  5.79,11.07 270 top
C43  24.1,5.26 270 top
C44  14.83,6.76 90 top
C51  23.22,30.05 180 top
C52  20.45,36.14 180 top
C53  24.08,36.14 0 top
CHARGING  2.59,30.84 180 top
D1  49.78,2.79 180 top
D4  5.73,38.67 270 top
D5  18.09,40.51 90 top
D31  10.95,23.29 180 top
D41  4.5,14.17 180 top
D42  18.44,4.55 90 top
D53  20.07,31.62 270 top
DISPLAY  50.37,50.16 0 top
E-FUSE-SWITCH  2.24,7.59 270 top
ESD_D1  35.74,4.5 180 top
FAULT  25.96,11.58 90 top
FLASHLIGHT  42.34,51.41 0 top
GND  32.77,33.02 0 top
GND1  27.69,38.1 70 top
GND2  27.69,25.4 70 top
GND3  27.69,17.78 70 top
GND4  27.69,33.02 70 top
I-SENSE-HEADER  64.24,49.02 270 top
IC1-BATT-PROTECT  6.74,44.87 90 top
IC2-CHARGER  11.04,38.52 270 top
IC3  8.71,27.86 90 top
IC4-E-FUSE  10.3,9.77 0 top
IC5-5V  23.32,33.12 90 top
IC6-I-SENSE  59.79,49.02 0 bottom
ICSP  41.94,42.19 0 top
ILIMIT  19.05,11.61 0 top
L31  14.63,29.21 0 top
LOGIC-PROBE  42.42,4.32 0 top
POW-SW  27.69,30.48 70 top
POW~12V  4.32,3.56 0 top
PWR-EN  32.77,30.48 0 top
R1  9.94,50.67 90 top
R2  15.73,44 90 top
R3  2.62,25.3 0 top
R4  36.3,41.15 0 top
R5  36.3,39.52 180 top
R6  48.69,22.89 225 top
R7  36.73,44.75 90 top
R8  44.2,48.26 90 top
R9  44.2,23.29 225 top
R10  39.65,23.85 225 top
R11  44.6,18.87 225 top
R12  39.83,19 225 top
R13  35.33,19.53 225 top
R14  16,36.07 90 top
R15  64.52,26.16 180 top
R16  60.96,23.06 90 top
R17  36.73,28.5 0 top
R18  35.76,25.88 180 top
R19  57.63,23.06 90 top
R20  48.26,44.2 180 top
R21  2.59,29.18 0 top
R22  2.62,32.91 180 top
R23  52.15,44.53 180 top
R24  53.64,46.69 180 top
R25  46.48,7.47 180 top
R26  46.25,4.83 90 top
R27  62.48,32.77 270 top
R28  49.91,46.66 0 top
R29  54.84,22.12 180 top
R30  59.28,23.06 90 top
R31  9.58,14.73 270 top
R32  3.45,18.08 270 top
R33  3.45,21.87 270 top
R34  12.47,15.7 180 top
R35  19.33,20.12 270 top
R36  64.52,12.09 270 top
R37  66.57,12.09 270 top
R38  10.67,44.2 90 top
R41  5.79,7.44 270 top
R42  4.22,8.31 270 top
R43  12.9,13.82 0 top
R46  9.88,2.69 90 top
R47  4.83,1.65 0 top
R48  25.96,15.14 90 top
RD1  24.46,43.43 90 top
RD2  22.78,43.43 90 top
RILIM1  16.69,13.89 180 top
RILIM2  20.35,13.94 0 top
RISET  9.81,35.06 0 top
ROTARY-ENCODER  56.16,10.34 180 top
S1  2.29,42.3 270 top
S2  13.11,44.34 270 top
S3  65.56,16.41 0 top
S4  15.21,40.38 90 top
S6  40.72,48.03 90 top
TP1  35.56,10.31 300 top
TP2  39.88,10.67 270 top
TP3  44.2,10.31 240 top
TVS_D2  36.86,33.73 270 top
U1  50.55,32.77 180 top
USB-ON  2.62,34.62 0 top
USBC  22.87,50.19 180 top
VBOOST  27.69,27.94 70 top
VBOOST-SEL  9.07,19.63 0 top
VIN  27.69,40.64 70 top
VIN'  32.77,40.64 0 top
VIN-ON  2.62,27 180 top
VOUT  27.69,20.32 70 top
VOUT'  32.77,20.32 0 top
VREF_SHUNT  65.28,30.23 0 top

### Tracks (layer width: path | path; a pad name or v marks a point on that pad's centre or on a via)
5V  (via drill 0.3)
  Top 0.406: R23.2 51.15,44.91 52.65,46.41 R24.2 | R28.2 51.15,46.42 R23.2 | R23.2 50.21,45.47 40.64,45.47 39.4,44.22 ICSP.VCC | R30.2 R19.2 57.63,24.61 v58.42,25.4 | R27.1 63.85,33.77 64.87,32.74 65.81,32.74 67.31,31.24 67.31,27.96 R15.1 66.08,25.6 v66.77,25.6 | R20.1 49.59,44.53 R23.2 | v33.48,14.09 32.26,12.87 32.26,5.16 32.92,4.5 | ESD_D1.5 32.92,4.5 | C12.1 32.92,2.5 32.92,4.5
  Top 0.508: 59.64,33.82 C4.1 62.41,33.84 R27.1 | D53.A 20.56,34.29 | 22.37,34.29 IC5-5V.5 22.09,34.7 | C52.2 19.45,35.24 | v35.05,43.18 35.2,43.33 R7.1 36.85,43.46 ICSP.VCC
  Top 0.559: C8.2 42.29,35.34 44.67,35.34 45.24,34.77 U1.18 47.35,34.77 48.72,33.39 52.58,33.39 | 59.64,33.82 C9.1 56.98,33.97 U1.6 53.55,33.97 52.97,33.39 52.58,33.39 | 52.58,33.39 53.6,32.37 U1.4
  Top 0.61: 20.56,34.29 22.37,34.29 | 22.09,34.7 19.98,34.7 19.45,35.24
  Top 0.813: C8.2 41.58,35.04 C10.1 38.99,35.92 TVS_D2.C 36.49,35.56 5V.P$1 5V-0.2A.P$1 27.94,35.64 25.78,37.8 20.8,37.8 19.45,36.44 C52.2 | D53.A 19.5,34.24
  Top 1.016: 19.5,34.24 19.5,36.09 C52.2
  Bottom 0.406: v58.42,25.4 66.57,25.4 v66.77,25.6 66.77,27.71 60.45,34.04 60.45,45.47 59.69,46.23 59.69,50.04 58.8,50.93 IC6-I-SENSE.8 | 5V.P$1 34.29,35.56 34.92,34.92 34.92,28.02 36.07,26.87 36.07,16.68 v33.48,14.09
  Bottom 0.508: v35.05,43.18 35.05,36.07 34.54,35.56 5V.P$1
  Bottom 0.813: 5V-0.2A.P$1 5V.P$1
!FLT  (via drill 0.3)
  Top 0.406: v19.13,9.78 19.1,9.78 18.46,9.13 IC4-E-FUSE.6 | FAULT.C v25.96,9.32
  Bottom 0.406: v19.13,9.78 25.5,9.78 v25.96,9.32
+VE
  Top 0.406: LOGIC-PROBE.1 43.18,6.35 44.36,6.35 R25.2
A
  Top 0.406: ROTARY-ENCODER.A 59.28,19.42 R30.1 R16.1
AREF
  Top 0.406: U1.20 44.14,33.17 43.61,33.69 C13.1
B
  Top 0.406: ROTARY-ENCODER.B 53.62,19.33 55.84,21.55 R29.1 55.9,22.06 R19.1
BATT+  (via drill 0.3)
  Top 0.406: v2.85,28.17 2.85,28.21 3.59,28.95 R21.2
  Top 0.61: 12.85,41.25 13.11,41.5 S2.5 13.11,41.38 v13.87,41.38 | 11.2,41.25 11.04,41.09 IC2-CHARGER.2
  Top 1.016: S4.3 13.87,40.76 v13.87,41.38 | v13.87,41.38 13.74,41.25 13.38,41.25 | 13.38,41.25 12.85,41.25 11.2,41.25 | S4.3 13.38,41.25 | v13.87,41.38 14.25,41 S4.3
  Bottom 0.406: v13.87,41.38 12.78,41.38 7.49,36.09 7.49,35.59 5.44,33.53 3.81,33.53 2.54,32.26 2.54,28.47 v2.85,28.17
BATT-
  Top 0.406: 6.1,45.53 6.74,44.9 IC1-BATT-PROTECT.9 7.43,45.56 8.64,45.56
  Top 1.016: 6.04,49.88 C1.2 | C1.2 5.71,49.5 5.71,47.96 IC1-BATT-PROTECT.7 | IC1-BATT-PROTECT.8 4.83,47.42 5.44,46.81 6.1,47.47 IC1-BATT-PROTECT.7 | 6.59,45.26 6.1,45.26 6.1,45.53 | IC1-BATT-PROTECT.7 6.1,45.53 | 6.1,45.53 IC1-BATT-PROTECT.13 | IC1-BATT-PROTECT.11 4.83,45.56 IC1-BATT-PROTECT.8 | IC1-BATT-PROTECT.8 4.83,49.88 C1.2 | IC1-BATT-PROTECT.5 8.64,45.56 IC1-BATT-PROTECT.17 | IC1-BATT-PROTECT.9 7.13,45.26
  Top 1.27: BATT_PORT.N 4.83,45.56
  Top 1.524: BATT_PORT.N 4.83,49.88
  Bottom 1.016: BATT_PORT.N 4.79,49.18 IC1-BATT-PROTECT.11 | IC1-BATT-PROTECT.11 IC1-BATT-PROTECT.13 | IC1-BATT-PROTECT.13 IC1-BATT-PROTECT.15 | IC1-BATT-PROTECT.15 IC1-BATT-PROTECT.17 IC1-BATT-PROTECT.16 IC1-BATT-PROTECT.14 | IC1-BATT-PROTECT.14 IC1-BATT-PROTECT.15 | IC1-BATT-PROTECT.14 IC1-BATT-PROTECT.12 | IC1-BATT-PROTECT.12 IC1-BATT-PROTECT.10 IC1-BATT-PROTECT.11 | IC1-BATT-PROTECT.13 IC1-BATT-PROTECT.12
  pour Bottom (no thermals): -0.2,54.15 -0.2,36.25 4.27,36.25 10.77,42.75 17.91,42.75 18.06,42.9 18.06,45.26 16.46,45.26 12.37,49.35 12.37,54.36 0,54.36
BATT_EN  (via drill 0.3)
  Top 0.406: D4.3 6.7,37.98 4.88,36.16 v4.88,36.02 | S2.3 11.11,45.64 R38.2 10.41,45.45 v10.41,46.43
  Bottom 0.406: v10.41,46.43 11.51,45.34 11.51,43.28 4.88,36.65 v4.88,36.02
BATTP_ALWAYS_ON
  Top 0.508: BATT_PORT.P 2.08,46.51 S1.1 | BATT+ON.P$1 BATT+ON'.P$1
  Top 0.61: S2.2 13.11,47.07 C2.2 | C2.2 13.64,47.29 13.69,47.24 13.69,45.85 13.9,45.64 S2.1 14.06,45.44 13.98,45.36 13.3,45.36 13.3,47.27 C2.2
  Top 1.016: R1.2 | 3.51,51.66 2.06,51 | BATT_PORT.P 2.75,51.46 2.84,51.66
  Top 1.27: 2.06,51.08 2.44,51.46 2.75,51.46 | 2.84,51.66 3.51,51.66 R1.2 | R1.2 10.97,51.67 11.84,50.8 11.84,48.78 C2.2
  Top 1.524: BATT_PORT.P 2.06,49.91 2.06,51 2.06,51.08
  Bottom 0.406: BATT+ON'.P$1 32.77,43.94 33.91,45.09 35.69,45.09 36.73,44.04 36.73,32.51 38.02,31.22 38.02,17.6 42.14,13.49 42.14,10.01 45.39,8.03 49.53,8.03 53.62,3.94 ROTARY-ENCODER.2
  Bottom 0.508: BATT_PORT.P 2.08,51.42 2.67,52 11.3,52 12.37,50.94 12.37,49.61 16.64,45.34 17.8,45.34 19.96,43.18 23.62,43.18 25.15,44.7 26.16,44.7 BATT+ON.P$1 BATT+ON'.P$1
BJT-B
  Top 0.406: R36.1 64.52,15.36 S3.1
BUZZER
  Top 0.508: U1.2 54.75,30.73 55.88,30.73 57.75,28.86 BUZZER.P$1
BYP1
  Top 0.61: IC5-5V.4 25.08,35.23 C53.2
CHG  (via drill 0.3)
  Top 0.406: IC2-CHARGER.3 10.09,38.86 10.41,38.53 12.45,38.53 12.6,38.37 13.76,38.37 v13.84,38.46 | CHARGING.C 4.1,30.84 4.62,31.36 v4.62,31.6
  Bottom 0.406: v13.84,38.46 11.71,38.46 5.33,32.08 5.11,32.08 v4.62,31.6
DISPLAY_VCC
  Top 0.406: R28.1 48.91,48.38 49.1,48.56 DISPLAY.VCC 49.1,49.15 49.84,49.89 49.84,50.9 C5.1
DVDT
  Top 0.406: C42.2 6.12,10.4 IC4-E-FUSE.2
EN/UVLO
  Top 0.406: IC4-E-FUSE.3 6.54,9.13 5.85,8.44 R41.1 5.49,8.44 4.35,7.31 R42.2
ENC_A
  Top 0.406: C17.1 61.49,19.36 62.1,19.97 62.1,23.55 61.59,24.06 R16.2 60.96,25.4 59.94,26.42 55.53,26.42 U1.32
ENC_B
  Top 0.406: U1.31 52.55,27.72 54.33,25.93 54.33,23.3 53.84,22.81 R29.2 53.84,21.58 51.66,19.41 C16.1
FB
  Top 0.406: 10.97,25.15 10.97,21.54
  Top 0.508: R31.1 9.58,19.13 VBOOST-SEL.C 10.97,21.54 | IC3.3 10.97,25.25 10.97,25.15
FL+
  Top 0.508: FLASHLIGHT.+VE 38.28,49.89 38.28,48.99 36.73,47.44 R7.2
FL-
  Top 0.508: S6.3 39.76,49.03 42.14,51.41 FLASHLIGHT.-VE
FLASHLIGHT_SIGNAL  (via drill 0.3)
  Top 0.305: 53.34,35.81 53.35,35.82
  Top 0.406: S6.1 44.02,47.08 R8.1 44.45,47.01 46.72,47.01 v47.15,46.58 | v48.42,35.01 48.81,34.62 52.15,34.62 53.34,35.81 | 53.35,35.82 U1.9
  Bottom 0.406: v47.15,46.58 47.24,46.58 47.97,45.85 47.97,35.47 v48.42,35.01
GND  (via drill 0.3, 0.35)
  Top 0.305: C4.2 60.33,31.84 61.25,32.77 63.39,32.77 64.97,31.19 VREF_SHUNT.3 | ESD_D1.2 36.3,4.5 36.19,4.46 35.52,2.11 C12.2 | S3.2 66.51,15.91 65.13,16.43 61.62,17.11 C17.2
  Top 0.406: R22.1 3.72,33.01 6.21,33.01 6.55,32.66 C31.1 | C5.2 47.5,51.09 46.83,50.42 46.83,49.67 46.56,49.4 DISPLAY.GND 46.19,49.26 R8.2 43.92,48.98 S6.2 | C14.1 C15.1 | VREF_SHUNT.2 66.03,29.47 66.03,30.11 65.28,30.86 VREF_SHUNT.3 | ROTARY-ENCODER.C 57.76,17.24 C17.2 | ESD_D1.2 38.86,4.5 40.39,2.97 42.34,2.97 LOGIC-PROBE.2 44.18,3.83 R26.1 | POW~12V.C 2.9,2.58 R47.1 2.67,1.65 v2.54,1.52 | R5.2 35.3,38.62 35.93,37.98 v37.8,37.98 | VIN-ON.C 4.85,27 v5.89,28.04 | R37.1 66.57,15.38 S3.2
  Top 0.508: S1.2 2.29,43.17 3.3,42.17 IC1-BATT-PROTECT.1 | 59.64,31.82 C4.2 | 56.87,31.57 C9.2 | v50.29,5.59 50.32,5.61 50.32,12.96 51.66,14.31 C16.2 54.37,17.03 ROTARY-ENCODER.C | 5.89,25.6 C6.1 | 15.73,46.89 C2.1 | RD1.1 25.86,42.43 | RD1.1 RD2.1 | R17.1 35.73,29.68 v35.84,29.79 35.84,30.52 TVS_D2.A | C7.1 C3.1 | C7.1 59.62,49.04 C15.1 | v56.64,45.97 56.6,46.02 C7.1 | RD1.1 25.89,42.43 v25.91,42.42
  Top 0.559: U1.5 55.77,33.17 C9.2 59.64,31.82 | 56.87,31.57 U1.3 53.02,31.57 52.22,32.37 U1.21 44.56,32.37 43.88,31.69 C13.2
  Top 0.61: IC2-CHARGER.5 11.04,35.28 10.83,35.08 | IC3.2 8.71,25.38 8.38,25.04 6.45,25.04 5.89,25.6 | C51.1 23.32,30.95 IC5-5V.2 23.32,33.12 | GND2.P$1 27.1,25.4 26.21,26.29 26.21,32.16 25.25,33.12 | RILIM1.1 18.54,14.75 | 18.54,14.75 v18.54,15.16 | RILIM2.1 18.54,14.75 | 23.32,33.12 25.25,33.12 | 25.25,33.12 27.84,33.12 GND4.P$1 | R2.2 15.73,46.89 | 23.32,33.12 23.32,35.91 C53.1 C52.1 | S2.4 12,43.2 R38.1 10.91,43.2 11.43,42.67 11.79,42.67 S2.4
  Top 0.711: R38.1 11.24,43.2 12.39,44.35 14.85,44.35 15.5,45 R2.2
  Top 0.762: 6.55,33.22 6.81,33.48
  Top 0.813: C13.2 42.93,31.69 C8.1 40.08,32.83 C10.2 38.59,33.04 v38.35,33.27 38.35,33.04 TVS_D2.A 35.38,33.02 GND.P$1 GND4.P$1 | GND1.P$1 27.71,38.1 26.19,39.62 25.86,39.62 | 25.86,39.62 25.86,42.43 25.86,45.52 25.62,45.75 USBC.B12 25.62,49.56 v24.13,51.05 v21.59,51.05 21.34,51.05 20.12,49.84 USBC.A12 20.12,46.36 18.97,45.21 15.94,45.21 R2.2 | R14.1 16.13,35.07 20.68,39.62 25.86,39.62 | IC4-E-FUSE.11 10.96,12.87 R43.1 11.82,13.73 R31.2 9.36,13.73 v8.53,14.55 7.98,15.11 v7.98,15.57 v7.14,15.6 6.7,15.16 D41.A 6.7,12.98 C42.1 | C41.1 5.71,11.99 C42.1 | C42.1 7.21,12.07 IC4-E-FUSE.1 9.61,11.68 IC4-E-FUSE.10 | IC1-BATT-PROTECT.4 9.64,42.17 R38.1
  Top 1.016: IC4-E-FUSE.9 IC4-E-FUSE.14 | 10.3,8.47 IC4-E-FUSE.16 | 11.1,5.92 11.26,5.76 C44.1 14.99,5.92 15.37,5.92 | v10.97,33.83 v12.24,33.83 v12.24,35.1 14.15,35.1 C21.1 R14.1
  Top 1.27: IC1-BATT-PROTECT.1 IC1-BATT-PROTECT.2 IC1-BATT-PROTECT.3 IC1-BATT-PROTECT.4 | 10.83,35.08 RISET.2 | 6.81,33.48 10.62,33.48 v10.97,33.83 10.83,33.98 10.83,35.08 | v12.24,35.1 10.86,35.1 10.83,35.08
  Top 1.524: IC1-BATT-PROTECT.4 8.44,41.97 8.44,37.4 6.55,35.51 C31.1 | C31.1 6.55,33.22 | C31.1 6.55,30.63 6.27,30.35 6.27,28.42 v5.89,28.04 6.17,27.76 v6.17,27.1 5.92,26.85 5.92,25.75 C6.1 | GND3.P$1 28.23,17.78 28.23,2.07 24.79,2.07 C43.2 23.69,2.34 D42.A 17.35,3.43 17.35,3.94 15.37,5.92 11.1,5.92 10.3,6.71 10.3,8.47 IC4-E-FUSE.15
  Bottom 0.406: v2.54,1.52 4.06,1.52 9.65,7.12 IC4-E-FUSE.16
  Bottom 0.508: IC4-E-FUSE.11 11.18,11.49 14.03,11.49 17.7,15.16 v18.54,15.16 | v38.35,33.27 37.8,33.83 v37.8,37.98 37.8,44.65 38.35,45.21 42.72,45.21 ICSP.GND 44.48,48.28 45.09,48.9 DISPLAY.GND 46.61,48.9 48.39,47.12 IC6-I-SENSE.5 56.64,46.67 v56.64,45.97 | ROTARY-ENCODER.C 56.16,18.82 55.75,19.23 BUZZER.P$2 | 36.83,29.23 36.83,12.63 37.8,10.16 38.86,6.22 42.05,6.22 43.69,4.59 LOGIC-PROBE.2 44.96,5.59 v50.29,5.59
  Bottom 0.61: v35.84,29.79 36.27,29.79 36.83,29.23
  Bottom 0.813: GND4.P$1 GND.P$1
  Bottom 1.016: 6.6,27.69 6.6,28.19 6.6,28.55 v6.5,28.65 v5.89,28.04 6.17,27.76 v6.17,27.1 6.68,27.61 6.6,27.69 | 6.6,27.69 6.35,27.94 | 11.94,33.53 11.63,33.83 v10.97,33.83 v12.24,35.1 v12.24,33.83 | 20.71,21.45 23.29,18.87 26.52,18.87 27.61,17.78 GND3.P$1
  Bottom 1.27: v7.98,15.57 8.48,15.06 8.48,14.58 8.15,14.58 v7.14,15.6
  Bottom 1.524: v7.14,15.6 7.11,15.57 4.65,18.03 4.65,22.68 6.35,24.38 6.35,27.94 | v7.98,15.57 8.91,16.51 15.77,16.51 20.71,21.45 24.66,25.4 GND2.P$1 | IC4-E-FUSE.14 IC4-E-FUSE.16 IC4-E-FUSE.17 IC4-E-FUSE.15 | IC4-E-FUSE.14 IC4-E-FUSE.15 | IC4-E-FUSE.15 IC4-E-FUSE.13 | IC4-E-FUSE.13 IC4-E-FUSE.11 IC4-E-FUSE.10 IC4-E-FUSE.12 | IC4-E-FUSE.12 IC4-E-FUSE.13 | IC4-E-FUSE.12 IC4-E-FUSE.14 | v12.24,33.83 11.94,33.53 11.94,31.75 12.7,30.99 12.7,29.46 11.43,28.19 6.6,28.19
  other vias: 31.5,14.81 33.78,16.76 37.59,14.48 43.18,14.48 46.48,14.48 48.77,14.48 20.07,49.78 25.65,49.28
  pour Bottom: 29.21,54.36 29.21,-1.27 28.96,-1.52 -0.51,-1.52 -1.02,-1.02 -1.02,35.87 4.35,35.87 10.72,42.24 18.62,42.24 18.84,42.46 18.9,45.75 16.81,45.8 12.88,49.73 12.88,54.36
  pour Bottom: 31.17,54.13 31.17,0.33 32.51,-1.02 68.58,-1.02 69.34,-0.25 69.34,52.83 68.05,54.13
  pour Top (no thermals): 3.81,12.19 4.32,12.19 5.33,13.21 5.33,14.99 6.35,14.99 6.6,15.24 7.87,15.24 7.87,14.99 8.64,14.22 12.19,14.22 12.19,13.21 11.94,12.95 11.33,12.95 11.33,11.58 3.81,11.58
  pour Top: 31.5,17.02 31.5,14.48 49.78,14.48 49.78,17.02
  pour Top: 31.5,17.02 31.5,14.22 50.04,14.22 50.04,17.02
I2C-SCL
  Top 0.305: 52.15,48.9 53.62,47.42 53.62,45
  Top 0.406: 52.15,48.9 DISPLAY.SCK 51.64,49.61 53.59,51.56 C14.2 | 53.62,45 R23.1 52.89,44.27 52.89,41.97 51.75,40.82 U1.11
I2C-SDA
  Top 0.406: C15.2 55.19,49.91 DISPLAY.SDA 54.65,48.43 R24.1 55.41,45.92 55.41,43.22 52.55,40.35 U1.10
I_MEASURE  (via drill 0.3)
  Top 0.406: U1.22 51.75,31.57 v52.58,30.73
  Bottom 0.406: v52.58,30.73 52.58,35.05 59.21,41.68 59.21,44.32 58.59,44.94 58.59,49.3 58.23,49.66 IC6-I-SENSE.7
ILM
  Top 0.508: ILIMIT.2 17.7,10.25 14.96,10.25 14.81,10.4 IC4-E-FUSE.7
ILM1
  Top 0.508: ILIMIT.1 15.69,12.43 RILIM1.2
ILM2
  Top 0.508: RILIM2.2 21.34,11.85 ILIMIT.3
IN+
  Bottom 0.762: IC6-I-SENSE.1 63.6,50.93 I-SENSE-HEADER.1 63.6,49.66 IC6-I-SENSE.2 IC6-I-SENSE.1
IN-
  Bottom 0.762: IC6-I-SENSE.3 63.6,48.39 I-SENSE-HEADER.2 63.6,47.12 IC6-I-SENSE.4 IC6-I-SENSE.3
ISET
  Top 0.61: RISET.1 8.81,35.23 10.09,36.5 IC2-CHARGER.4
N$1
  Top 0.406: USBC.B5 22.37,45.7 22.86,45.21 22.86,44.51 RD2.2
N$2
  Top 0.406: USBC.A5 23.37,46.33 24.46,45.24 RD1.2
N$3
  Top 0.406: USB-ON.C R22.2
N$4
  Top 0.508: R32.2 3.79,17.1 6.33,19.63 VBOOST-SEL.1
N$5
  Top 0.406: R3.1 VIN-ON.A
N$7
  Top 0.406: R48.1 FAULT.A
N$10
  Top 0.406: CHARGING.A R21.1
N$12
  Top 0.508: R32.1 R33.2
N$13
  Top 0.508: R34.2 11.47,19.5 VBOOST-SEL.2
N$18
  Top 0.406: POW~12V.A 5.83,3.47 R47.2 9.84,1.65 R46.1
N$21
  Top 0.406: R34.1 15.76,17.98 17.42,17.98 19.33,19.89 R35.3
OVLO  (via drill 0.3)
  Top 0.406: R42.1
  Top 0.508: v3.94,10.44 3.94,9.59 R42.1 | IC4-E-FUSE.8 13.01,12.09 v13.51,12.6 13.9,12.99 R43.2
  Bottom 0.406: v3.94,10.44 6.68,13.18 12.93,13.18 v13.51,12.6
POWER_EN_SOFT  (via drill 0.3)
  Top 0.406: v48.44,1.45 49.45,1.45 49.45,1.5 D1.3
  Top 0.508: POW-SW.P$1 PWR-EN.P$1
  Bottom 0.406: PWR-EN.P$1 33.07,30.18 33.07,27.64 34.47,26.24 34.47,19.3 32.49,17.32 32.49,3.46 34.71,1.24 48.23,1.24 v48.44,1.45
  Bottom 0.508: S1.3 1.29,37.31 1.29,27.96 2.13,27.13 3.33,27.13 3.86,27.66 3.86,29.62 5.16,30.91 6.3,30.91 11.96,36.58 13.46,36.58 14.22,35.81 14.22,32 15.75,30.48 POW-SW.P$1 PWR-EN.P$1
POWER_EN_TB
  Top 0.305: D1.2 49,3.75 50.27,2.77 51.4,2.35
  Top 0.508: R37.2 R36.2 64.35,11.09 62.33,9.07 62.33,6.43 58.7,2.79 ROTARY-ENCODER.1 58.7,2.52 57.67,3.56 52.6,3.56 51.4,2.35
PWR_CTRL
  Top 0.406: U1.30 51.75,27.25 53.49,25.5 53.49,24.64 52.6,23.75 52.6,21.82 50.06,19.28 50.06,14.25 49.02,13.21 49.02,5.47 D1.1
PWR_SW
  Top 0.406: D4.1 4.27,40.13 2.47,40.13 S1.C
RESET  (via drill 0.3)
  Top 0.406: ICSP.RESET 47.26,43.7 R20.2 47.26,43.94 48.28,42.93 51.56,42.93 v51.82,42.67 | v51.31,30.73 50.95,30.37 U1.29
  Bottom 0.406: v51.82,42.67 51.56,42.42 51.56,30.99 v51.31,30.73
RT
  Top 0.406: R2.1 15.69,43.04 S2.6
SW
  Top 0.61: IC3.1 7.76,27.61 8.02,27.86 12.78,27.86
  Top 1.27: 12.78,27.86 L31.P$2 13.15,24.53 D31.A
TEST_BUTTON
  Top 0.406: U1.1 57.25,27.43 62.25,27.43 R15.2 63.52,23.67 62.86,23.02 62.86,20.06 S3.3
TP1
  Top 0.406: R10.2 39.48,22.01 39.48,21.14 | 39.48,21.14 43.28,24.94 43.28,26.64 46.38,29.74 U1.24 | ESD_D1.4 34.44,6.6 35.95,8.11 TP1.3 | 39.48,21.14 35.56,17.22
  Top 0.508: TP1.3 TP1.2 TP1.1 35.56,13.78 35.56,17.22 35.56,17.29 R13.2
TP1_470K/SCK  (via drill 0.3)
  Top 0.406: R13.1 36.29,20.59 36.29,23.1 40.36,27.18 v40.89,27.18 | U1.17 46.05,35.57 45.16,36.45 41.05,36.45 v40.92,36.58
  Bottom 0.406: ICSP.SCK 40.92,39.9 v40.92,36.58 40.92,27.2 v40.89,27.18
TP1_680/MISO  (via drill 0.3)
  Top 0.406: U1.16 46.22,38.46 41.85,38.46 ICSP.MISO | v39.42,27.79 39.95,28.32 41.55,28.32 42.08,27.8 42.08,26.28 R10.1
  Bottom 0.406: ICSP.MISO 39.42,40.89 v39.42,27.79
TP2
  Top 0.305: 38.38,6.63 36.25,6.63 35.85,6.3 35.34,3.55 ESD_D1.6
  Top 0.406: R9.2 43.95,21.52 43.95,20.66 | 43.95,20.66 47.14,23.85 47.14,27.99 U1.25 | 38.38,6.63 TP2.3 | 43.95,20.66 39.88,16.59
  Top 0.508: TP2.3 TP2.2 TP2.1 39.88,16.59 39.88,16.94 R12.2
TP2_470K/MOSI  (via drill 0.3)
  Top 0.406: U1.15 48.55,38.37 47.52,39.4 43.69,39.4 43.2,39.88 43.2,42.19 ICSP.MOSI | v42.22,20.57 42.22,20.52 41.7,20 R12.1
  Bottom 0.406: ICSP.MOSI 43.2,42.19 43.2,21.49 42.29,20.57 v42.22,20.57
TP2_680/SIGNAL_OUT  (via drill 0.3)
  Top 0.406: v45.34,26.31 45.2,26.18 R9.1 | v46.74,40.89 47.75,40.89 49.35,39.3 U1.14
  Bottom 0.406: v46.74,40.89 46.74,27.71 v45.34,26.31
TP3
  Top 0.406: U1.26 48.55,26.61 48.01,26.07 48.01,22.2 R6.2 48.22,21.35 48.22,18.6 47.14,17.53 44.45,17.53 | TP3.3 42.15,8.11 39.47,5.44 37.05,5.44 ESD_D1.3
  Top 0.508: TP3.3 TP3.2 TP3.1 45.47,16.51 44.45,17.53 44.11,17.87 R11.2
TP3_470K  (via drill 0.3)
  Top 0.406: R11.1 46.69,18.8 v47.02,18.8 | v49.05,41.35 50.15,40.25 U1.13
  Bottom 0.406: v47.02,18.8 49.3,21.08 49.3,41.1 v49.05,41.35
TP3_680  (via drill 0.3)
  Top 0.406: R6.1 50.47,24.66 v50.47,25.15 | v50.29,41.91 50.95,41.26 U1.12
  Bottom 0.406: v50.29,41.91 50.39,41.91 50.47,41.83 v50.47,25.15
TP_LOGIC
  Top 0.406: U1.27 49.35,26.85 50.22,25.98 50.72,25.98 51.51,25.2 51.51,24.51 51.71,24.3 51.71,22.5 49.17,19.96 49.17,17.68 47.74,16.24 47.74,7.72 R25.1 47.48,7.05 R26.2 46.46,5.83 47.62,4.66 47.62,2.62 47.19,2.18 39.4,2.18 38.03,3.55 ESD_D1.1
TS  (via drill 0.3)
  Top 0.406: IC2-CHARGER.1 12.66,39.82 13.03,39.45 v13.16,39.45
USBV  (via drill 0.3)
  Top 0.406: D4.2 4.78,37.58 3.63,36.44 3.63,34.64 USB-ON.A 4.78,34.62 v4.83,34.67
  Top 0.61: IC2-CHARGER.6 12.03,37.18 12.19,37.18
  Top 0.762: 21.84,49.53 21.35,49.04 USBC.A9 21.35,45.62 v21.22,45.49 | v22.4,49.53 v23.37,49.53 23.88,49.53 24.39,49.02 USBC.B9 | 18.04,39.43 S4.1 16.42,39.17 16.42,38.6 v16.26,38.43 16.26,37.32 R14.2 16,37.23
  Top 0.813: 21.84,49.53 v22.4,49.53
  Top 1.016: 12.29,37.08 12.19,37.18 | 21.22,45.2 20.9,44.88 v20.7,44.88 | 21.22,45.2 v21.22,45.49 | v20.7,44.88 21.02,45.2 21.22,45.2 | v20.7,44.88 20.7,44.68 20.37,44.35 20.22,44.2 20.22,44.4 v20.7,44.88
  Top 1.27: 12.29,37.08 C21.2 14.18,37.07 R14.2 | 20.37,44.35 20.37,41.58 18.14,39.35 D5.A 18.04,39.43
  Top 1.524: D5.A 16,37.23
  Bottom 0.406: v4.83,34.67 5.13,34.67 6.1,35.64 6.1,36.32 12.45,42.67 14.99,42.67 16.26,41.4 v16.26,38.43
  Bottom 0.813: v20.7,44.88 21.31,45.49 | 21.31,45.49 21.39,45.57 21.51,45.57 22.86,46.91 22.86,49.53 | 22.86,49.53 v23.37,49.53 v22.4,49.53 22.86,49.53 | v21.22,45.49 21.31,45.49
  Bottom 1.016: v21.22,45.49 21.22,45.4 v20.7,44.88
VBATT_MEASURE  (via drill 0.3)
  Top 0.406: v44.78,37.54 41.43,37.54 39.45,39.52 R5.1 R4.2 | U1.19 44.83,33.97 44.76,34.04 v44.77,34.05
  Bottom 0.406: v44.77,34.05 v44.77,37.53 v44.78,37.54
VBOOST  (via drill 0.3)
  Top 0.61: 5.99,22.89 5.98,22.87 R33.1
  Top 1.016: D31.C 8.74,22.2 v9.22,21.72 | v9.22,21.72 8.26,21.72 v8.18,21.79 8.13,21.84 7.54,21.84 v7.29,21.59 5.99,22.89 | v9.22,21.72 9.22,23.19 9.4,23.37 8.82,23.37 8.34,22.89
  Top 1.473: R33.1 1.79,22.87 1.78,22.86 1.78,14.69 D41.C | 1.95,13.83 C41.2 1.93,11.97 1.93,9.17 E-FUSE-SWITCH.1
  Top 1.524: D31.C 8.34,22.89 5.99,22.89 C6.2 5.88,22.87 R33.1 | D41.C 1.95,13.83
  Bottom 0.508: 12.42,22.05 14.86,22.05 R35.2
  Bottom 1.524: VBOOST.P$1 25.53,27.94 24.82,28.65 19.02,28.65 12.42,22.05 10.46,22.05 10.41,22.1 9.6,22.1 v9.22,21.72 8.97,21.97 8.36,21.97 v8.18,21.79 7.49,21.79 v7.29,21.59
VBOOST2
  Top 0.406: R46.2 7.13,6.44 5.84,6.44
  Top 0.508: 7.87,7.87 7.61,7.87 IC4-E-FUSE.4 6.18,6.44 R41.2
  Top 1.016: R41.2 5.84,6.44
  Top 1.27: E-FUSE-SWITCH.2 2.29,6.27 2.29,5.59 6.1,5.59 6.1,6.19 5.84,6.44
  pour Top (no thermals): 6.86,8.13 8.36,8.13 8.36,5.13 8.23,5 0.28,5 0.28,6.6 1.85,6.6 2.57,5.89 5.13,5.77 6.88,7.52 6.86,7.52
VDD
  Top 0.61: C1.1 8.06,49.6 7.37,48.91 IC1-BATT-PROTECT.6
  Top 0.813: R1.1 8.25,49.67 C1.1
VIN  (via drill 0.3, 0.35)
  Top 0.406: v16.56,32 16.05,32 15.8,31.75 15.8,28.93 17.55,27.18 17.55,26.47 19.36,24.66 19.91,24.66 20.95,23.62 v20.95,18.85 | R4.1 33.27,41.15 VIN'.P$1 | R48.2 25.96,17.4 v25.93,17.42 | v2.95,24.23 2.95,24.63 R3.2 | v10.67,30.38 9.68,31.37 9.5,31.37
  Top 0.508: VIN.P$1 VIN'.P$1
  Top 0.61: C31.2 9.4,31.06 8.71,30.38 IC3.5 9,28.88 9.42,28.88 9.71,29.16 IC3.4 9.61,29.16
  Top 0.762: 9.61,29.16 9.5,29.28
  Top 1.016: v16.56,32 16.59,32 | 15.04,32 L31.P$1 | D5.C 17.8,41.33 S4.2 16.83,41.33 17.7,42.2 v17.7,42.93 | D5.C 18.54,42.07 v18.54,42.93 | v18.54,42.93 18.59,42.98 18.11,43.46 v18.11,43.64 18.11,43.33 v17.7,42.93 | v18.54,42.93 v17.7,42.93 | v17.7,42.93 18.12,42.51 D5.C
  Top 1.27: 16.59,32 v16.59,32.97 15.19,32.97 L31.P$1 13.95,31.73 9.65,31.73 C31.2 9.5,31.37 9.5,29.28 | v16.56,32 15.04,32
  Bottom 0.406: v25.93,17.42 22.45,17.42 21.03,18.85 v20.95,18.85 | v10.67,30.38 7.52,30.38 7.01,29.87 5.89,29.87 4.83,28.8 4.83,27.03 3.23,25.43
  Bottom 0.508: 3.23,25.43 3.23,24.51 v2.95,24.23 | VIN.P$1 VIN'.P$1
  Bottom 1.016: v16.59,32.97 16.59,32 v16.56,32 16.51,32 16,32.51 16,32.94 | v16.59,32.97 16.59,33.53 | 16.46,32.97 v16.59,32.97 | v16.59,32.97 17.02,32.54 | 17.02,32.54 17.02,32.44 | 17.02,32.54 17.02,33.1 | v18.54,42.93 18.11,43.36 v18.11,43.64 | v18.11,43.64 18.11,43.33 v17.7,42.93 18.16,42.93 18.54,42.55 v18.54,42.93 | v18.11,43.64 18.54,43.2 v18.54,42.93
  Bottom 1.27: 16.59,33.53 16.59,34.95 | 16,32.51 16.46,32.97 | 17.02,32.44 16.59,32 | 17.02,33.1 16.59,33.53 | 16,32.94 16.59,33.53
  Bottom 1.524: 16.59,34.95 16.59,35.64 18.54,37.59 18.54,40.64 | 18.54,40.64 18.54,42.55 | VIN.P$1 18.54,40.64
VIN5V  (via drill 0.3)
  Top 0.61: IC5-5V.3 24.82,31.82 25.09,31.55 v25.17,31.55 | IC5-5V.1 22.37,30.2 C51.2 | C51.2 22.22,30.72 v21.46,31.47 21.64,31.29 21.64,30.62 C51.2
  Top 1.016: C51.2 20.72,30.05 D53.K 20.01,26.93 5V-SWITCH.2
  Bottom 0.61: v25.17,31.55 21.54,31.55 v21.46,31.47
VOUT
  Top 0.406: VOUT'.P$1 34.76,22.32 R18.2
  Top 0.508: VOUT.P$1 VOUT'.P$1
  Top 1.016: 24.11,18.59 24.38,18.87 24.38,25.09 5V-SWITCH.1
  Top 1.524: C43.1 24.11,18.59 24.11,19.3 25.12,20.32 VOUT.P$1
  Bottom 0.508: VOUT.P$1 VOUT'.P$1
  pour Top (no thermals): 12.27,8.13 12.27,7.06 16.3,7.06 17.91,5.46 25.4,5.46 25.4,8.13
VOUT_MEASURE
  Top 0.406: R17.2 38.77,29.54 43.74,29.54 44.97,30.77 U1.23
  Top 0.508: R17.2 37.78,28.45 37.78,26.9 R18.1
VREF_2.5V  (via drill 0.3)
  Top 0.406: R27.2 62.48,31.44 64.33,29.59 VREF_SHUNT.1 63.83,28.77 v63.83,27.84 | U1.28 50.15,27.38 50.67,26.85 51,26.85 52.5,25.35 v52.5,25.25
  Bottom 0.406: v52.5,25.25 53.92,26.67 62.66,26.67 v63.83,27.84
XTAL1
  Top 0.406: 62.28,42.42 20MHZ.2
  Top 0.508: 20MHZ.2 62.28,44.34 C3.2 | U1.7 55.85,34.77 62.28,41.2 62.28,42.42
XTAL2
  Top 0.508: C7.2 57.4,44.82 20MHZ.1 57.4,38.25 U1.8

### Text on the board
tPlace: SW OFF ON | LIPO / CHARGE BOOST / PROTECT | VBOOST | 3.3V-17V | 5.5V | 3.3V-17V | 0.5A 1.6A | VOUT / 3V-16V | TRANSISTOR COMPONENT TESTER | TEST / BUTTON
bPlace: TS | v1

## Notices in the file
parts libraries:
SparkFun-PowerSymbols: Licensing: Creative Commons ShareAlike 4.0 International - https://creativecommons.org/licenses/by-sa/4.0
